|   Microchip Technology Inc.
|   PolarFire IBIS Model
[IBIS ver]   5.0
[File name]   polarfire_gpio_diff.ibs
[File Rev]   2.4
[Date]   Fri Nov 24 2023
[Source] Simulated Models ONLY.
   All data is based on Spice simulation. All performed at Microchip Technology Inc.
[Notes]   This IBIS file is for GPIO Differential Standards.
   Please refer to polarfire_gpio_se.ibs for GPIO single ended Standards Configurations,
   and refer to polarfire_hsio_se.ibs and polarfire_hsio_diff.ibs for HSIO Configurations.
   The package parasitics of various package types are given.
   Uncomment the appropriate package before simulations
   Revision History
   Rev 2.4: 24-Nov-2023
   - Added clamp-off configuration support for LCMDS25,SLVS25,LVDS25,PPDS25,RSDS25,SUBLVDS25,
   MINILVDS25,HCSL25 receivers
   - Added mixed mode receiver support for HSUL18_33_ODT-OFF,HSUL18_25_ODT-OFF,HSUL18_15_ODT-OFF,
   HSUL18_12_ODT-OFF,HSUL18_ODT-OFF,HSUL18_ODT-50
   - Updated Vinl and Vinh values of HCSL33, HCSL25 receivers
   Rev 2.3: 20-Jun-2023
   - Added VCM-LOW configuration support for SLVS33,SLVS25,LVDS33,LVDS25,RSDS33,RSDS25,
   MINILVDS33,MINILVDS25,SUBLVDS33,SUBLVDS25,PPDS33,PPDS25,HCSL33,HCSL25,LVPECL33,LVDS18G receivers
   - Updated Vmeas values of LCMDS33,LCMDS25,MIPIE25 drivers
   - Updated Vinl and Vinh values of SLVS33,SLVS25 receivers
   Rev 2.2: 4-May-2022
   - Added MPF050 device with RLC package data in [Package] section
   - Added RLC package type of FCG784N for MPF300T/TS device
   - Update RLC values of 200T-FCVG484 device package data
   Rev 2.1: 06-Sept-2021
   - Added support for LVDS18G driver and receiver
   - All LVDS type differential driver models updated to provide stable common mode voltage
[Disclaimer] This information is for board design considerations.
   Simulation based V/I curves contained in this model file are
   considered preliminary until verified against bench
   measurements. Maximum currents may vary from part to part but
   should not exceed maximum I/V curves provided in this model file.
[Copyright]  (c) 2023, Microchip Technology Inc., All Rights Reserved.
| ADDITIONAL NOTES
|For High Speed Mobile Industry Processor Interface (MIPI) configuration,please use LVDS25 receiver IBIS models.
|Warnings for ISSO Pullup, Pulldown currents being non-zero maybe ignored.
|Cautions for Ramp data maybe ignored.
|The naming conventions used in the signal_name/model_name are as follows:
| SLEW-#  - Slew setting,OFF or ON represented by #
| HYST-# and HYS-#  - Hysteresis setting,OFF or ON represented by #
| #mA   - Driver current strength, value represented by #
| #ohm   - Driver impedance mode, value represented by #
| ODT-# and OD-#   - Series on-die termination, impedance value represented by #
| CL   - Receiver standards with clamp ON
| C1   - Refers to Class-I driver models
| C2   - Refers to Class-II driver models
| #_I   - Refers to input models ,  model name represented by #
| #_O   - Refers to output models , model name represented by #
| VCML   - Refers to LOW Vcm setting
| VCMM   - Refers to MID Vcm setting
| IBIS MODEL CHECKLIST
| Microchip Technology Inc. is dedicated to releasing quality IBIS models to customers.
| The following items have been
| verified for this IBIS model before release:
| 1)  Checked IBIS model by the golden parser ibischk5 [Complete]
| 2)  Ensured no errors reported by golden parser
|   for the IBIS model [Complete]
| 3)  Defined Vinl and Vinh for receivers [Complete]
| 4)  Defined Standard Load and Vmeas values for drivers [Complete]
| 5)  Defined overshoots for drivers and receivers [NA]
| 6)  Validated Ramp Values[]
| 7)  Defined V-T Tables for all output drivers [Complete]
| 8)  Validated [Diff Pins] [Complete]
| 9)  Verified Package Parasitics [Complete]
| 10) Defined Standard Load Parameters and Specifications
|   for waveforms [Complete]
| 11) Defined and Validate Pin mappings [Complete]
| 12) Verified C_comp_pullup and C_comp_pulldown Values []
| 13) Visually Inspected I-V Curves and V-T Tables  [Complete]
| 14) Presented Typ/Min/Max Values in the correct order for
|   all tables and parameters [Complete]
| 15) Simulated all output models with standard load and
|   switching through Vmeas [Complete]
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[Component]   PolarFire
[Manufacturer]   Microchip Technology Inc
[Package]
|   typ   min   max
|MPF050T/TL/TLS/TS
|R_pkg   0.342   NA   NA   | MPF050T/TL/TLS/TS-FCSG325
|L_pkg   2.917nH   NA   NA   | MPF050T/TL/TLS/TS-FCSG325
|C_pkg   1.401pF   NA   NA   | MPF050T/TL/TLS/TS-FCSG325
|R_pkg   0.668   NA   NA   | MPF050T/TL/TLS/TS-FCVG484
|L_pkg   4.858nH   NA   NA   | MPF050T/TL/TLS/TS-FCVG484
|C_pkg   1.717pF   NA   NA   | MPF050T/TL/TLS/TS-FCVG484
|MPF100T/TL/TLS/TS
|R_pkg   0.277   NA   NA   | MPF100T/TL/TLS/TS-FCSG325
|L_pkg   2.866nH   NA   NA   | MPF100T/TL/TLS/TS-FCSG325
|C_pkg   0.601pF   NA   NA   | MPF100T/TL/TLS/TS-FCSG325
|R_pkg   0.960   NA   NA   | MPF100T/TL/TLS/TS-FCG484
|L_pkg   6.090nH   NA   NA   | MPF100T/TL/TLS/TS-FCG484
|C_pkg   2.182pF   NA   NA   | MPF100T/TL/TLS/TS-FCG484
|R_pkg   0.639   NA   NA   | MPF100T/TL/TLS/TS-FCVG484
|L_pkg   4.241nH   NA   NA   | MPF100T/TL/TLS/TS-FCVG484
|C_pkg   1.595pF   NA   NA   | MPF100T/TL/TLS/TS-FCVG484
|MPF200T/TL/TLS/TS
|R_pkg   0.392   NA   NA   | MPF200T/TL/TLS/TS-FCSG325
|L_pkg   3.035nH   NA   NA   | MPF200T/TL/TLS/TS-FCSG325
|C_pkg   0.970pF   NA   NA   | MPF200T/TL/TLS/TS-FCSG325
|R_pkg   0.885   NA   NA   | MPF200T/TL/TLS/TS-FCG484
|L_pkg   5.836nH   NA   NA   | MPF200T/TL/TLS/TS-FCG484
|C_pkg   2.013pF   NA   NA   | MPF200T/TL/TLS/TS-FCG484
|R_pkg   0.634   NA   NA   | MPF200T/TL/TLS/TS-FCVG484
|L_pkg   4.221nH   NA   NA   | MPF200T/TL/TLS/TS-FCVG484
|C_pkg   1.605pF   NA   NA   | MPF200T/TL/TLS/TS-FCVG484
|R_pkg   0.483   NA   NA   | MPF200T/TL/TLS/TS-FCSG536
|L_pkg   4.073nH   NA   NA   | MPF200T/TL/TLS/TS-FCSG536
|C_pkg   1.335pF   NA   NA   | MPF200T/TL/TLS/TS-FCSG536
|R_pkg   1.512   NA   NA   | MPF200T/TL/TLS/TS-FCG784
|L_pkg   9.182nH   NA   NA   | MPF200T/TL/TLS/TS-FCG784
|C_pkg   3.029pF   NA   NA   | MPF200T/TL/TLS/TS-FCG784
|MPF300T/TL/TLS/TS
|R_pkg   0.678   NA   NA   | MPF300T/TL/TLS/TS-FCG484
|L_pkg   5.038nH   NA   NA   | MPF300T/TL/TLS/TS-FCG484
|C_pkg   1.584pF   NA   NA   | MPF300T/TL/TLS/TS-FCG484
|R_pkg   0.702   NA   NA   | MPF300T/TL/TLS/TS-FCVG484
|L_pkg   4.503nH   NA   NA   | MPF300T/TL/TLS/TS-FCVG484
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R_pkg   1.478   NA   NA   | MPF300T/TL/TLS/TS-FCG1152
L_pkg   8.879nH   NA   NA   | MPF300T/TL/TLS/TS-FCG1152
C_pkg   2.839pF   NA   NA   | MPF300T/TL/TLS/TS-FCG1152
|MPF500T/TL/TLS/TS
|R_pkg   1.081   NA   NA   | MPF500T/TL/TLS/TS-FCG784
|L_pkg   6.727nH   NA   NA   | MPF500T/TL/TLS/TS-FCG784
|C_pkg   2.413pF   NA   NA   | MPF500T/TL/TLS/TS-FCG784
|R_pkg   1.419   NA   NA   | MPF500T/TL/TLS/TS-FCG1152
|L_pkg   8.917nH   NA   NA   | MPF500T/TL/TLS/TS-FCG1152
|C_pkg   2.924pF   NA   NA   | MPF500T/TL/TLS/TS-FCG1152
| End Header
| The PIN numbers given below are examples. They do not correspond to
| device pin numbers.
[Pin]   signal_name   model_name   R_pin   L_pin   C_pin
1N   SSTL25D_C1_80ohm_SLEW-OFF_N_O   SSTL25_C1_80ohm_SLEW-OFF_GPIO_O
1P   SSTL25D_C1_80ohm_SLEW-OFF_P_O   SSTL25_C1_80ohm_SLEW-OFF_GPIO_O
2N   SSTL25D_C1_120ohm_SLEW-OFF_N_O   SSTL25_C1_120ohm_SLEW-OFF_GPIO_O
2P   SSTL25D_C1_120ohm_SLEW-OFF_P_O   SSTL25_C1_120ohm_SLEW-OFF_GPIO_O
3N   SSTL25D_C1_60ohm_SLEW-OFF_N_O   SSTL25_C1_60ohm_SLEW-OFF_GPIO_O
3P   SSTL25D_C1_60ohm_SLEW-OFF_P_O   SSTL25_C1_60ohm_SLEW-OFF_GPIO_O
4N   SSTL25D_C1_48ohm_SLEW-OFF_N_O   SSTL25_C1_48ohm_SLEW-OFF_GPIO_O
4P   SSTL25D_C1_48ohm_SLEW-OFF_P_O   SSTL25_C1_48ohm_SLEW-OFF_GPIO_O
5N   SSTL25D_C2_48ohm_SLEW-OFF_N_O   SSTL25_C2_48ohm_SLEW-OFF_GPIO_O
5P   SSTL25D_C2_48ohm_SLEW-OFF_P_O   SSTL25_C2_48ohm_SLEW-OFF_GPIO_O
6N   SSTL25D_C2_60ohm_SLEW-OFF_N_O   SSTL25_C2_60ohm_SLEW-OFF_GPIO_O
6P   SSTL25D_C2_60ohm_SLEW-OFF_P_O   SSTL25_C2_60ohm_SLEW-OFF_GPIO_O
7N   SSTL25D_C2_40ohm_SLEW-OFF_N_O   SSTL25_C2_40ohm_SLEW-OFF_GPIO_O
7P   SSTL25D_C2_40ohm_SLEW-OFF_P_O   SSTL25_C2_40ohm_SLEW-OFF_GPIO_O
8N   SSTL25D_C2_34ohm_SLEW-OFF_N_O   SSTL25_C2_34ohm_SLEW-OFF_GPIO_O
8P   SSTL25D_C2_34ohm_SLEW-OFF_P_O   SSTL25_C2_34ohm_SLEW-OFF_GPIO_O
9N   SSTL18D_C1_60ohm_SLEW-OFF_N_O   SSTL18_C1_60ohm_SLEW-OFF_GPIO_O
9P   SSTL18D_C1_60ohm_SLEW-OFF_P_O   SSTL18_C1_60ohm_SLEW-OFF_GPIO_O
10N   SSTL18D_C1_80ohm_SLEW-OFF_N_O   SSTL18_C1_80ohm_SLEW-OFF_GPIO_O
10P   SSTL18D_C1_80ohm_SLEW-OFF_P_O   SSTL18_C1_80ohm_SLEW-OFF_GPIO_O
11N   SSTL18D_C1_48ohm_SLEW-OFF_N_O   SSTL18_C1_48ohm_SLEW-OFF_GPIO_O
11P   SSTL18D_C1_48ohm_SLEW-OFF_P_O   SSTL18_C1_48ohm_SLEW-OFF_GPIO_O
12N   SSTL18D_C1_40ohm_SLEW-OFF_N_O   SSTL18_C1_40ohm_SLEW-OFF_GPIO_O
12P   SSTL18D_C1_40ohm_SLEW-OFF_P_O   SSTL18_C1_40ohm_SLEW-OFF_GPIO_O
13N   SSTL18D_C2_40ohm_SLEW-OFF_N_O   SSTL18_C2_40ohm_SLEW-OFF_GPIO_O
13P   SSTL18D_C2_40ohm_SLEW-OFF_P_O   SSTL18_C2_40ohm_SLEW-OFF_GPIO_O
14N   SSTL18D_C2_48ohm_SLEW-OFF_N_O   SSTL18_C2_48ohm_SLEW-OFF_GPIO_O
14P   SSTL18D_C2_48ohm_SLEW-OFF_P_O   SSTL18_C2_48ohm_SLEW-OFF_GPIO_O
15N   SSTL18D_C2_34ohm_SLEW-OFF_N_O   SSTL18_C2_34ohm_SLEW-OFF_GPIO_O
15P   SSTL18D_C2_34ohm_SLEW-OFF_P_O   SSTL18_C2_34ohm_SLEW-OFF_GPIO_O
16N   SSTL18D_C2_30ohm_SLEW-OFF_N_O   SSTL18_C2_30ohm_SLEW-OFF_GPIO_O
16P   SSTL18D_C2_30ohm_SLEW-OFF_P_O   SSTL18_C2_30ohm_SLEW-OFF_GPIO_O
17N   SSTL15D_C1_40ohm_SLEW-OFF_N_O   SSTL15_C1_40ohm_SLEW-OFF_GPIO_O
17P   SSTL15D_C1_40ohm_SLEW-OFF_P_O   SSTL15_C1_40ohm_SLEW-OFF_GPIO_O
18N   SSTL15D_C1_48ohm_SLEW-OFF_N_O   SSTL15_C1_48ohm_SLEW-OFF_GPIO_O
18P   SSTL15D_C1_48ohm_SLEW-OFF_P_O   SSTL15_C1_48ohm_SLEW-OFF_GPIO_O
19N   SSTL15D_C2_34ohm_SLEW-OFF_N_O   SSTL15_C2_34ohm_SLEW-OFF_GPIO_O
19P   SSTL15D_C2_34ohm_SLEW-OFF_P_O   SSTL15_C2_34ohm_SLEW-OFF_GPIO_O
20N   SSTL15D_C2_30ohm_SLEW-OFF_N_O   SSTL15_C2_30ohm_SLEW-OFF_GPIO_O
20P   SSTL15D_C2_30ohm_SLEW-OFF_P_O   SSTL15_C2_30ohm_SLEW-OFF_GPIO_O
21N   SSTL15D_C2_27ohm_SLEW-OFF_N_O   SSTL15_C2_27ohm_SLEW-OFF_GPIO_O
21P   SSTL15D_C2_27ohm_SLEW-OFF_P_O   SSTL15_C2_27ohm_SLEW-OFF_GPIO_O
22N   HSUL18D_C1_55ohm_SLEW-OFF_N_O   HSUL18_C1_55ohm_SLEW-OFF_GPIO_O
22P   HSUL18D_C1_55ohm_SLEW-OFF_P_O   HSUL18_C1_55ohm_SLEW-OFF_GPIO_O
23N   HSUL18D_C1_60ohm_SLEW-OFF_N_O   HSUL18_C1_60ohm_SLEW-OFF_GPIO_O
23P   HSUL18D_C1_60ohm_SLEW-OFF_P_O   HSUL18_C1_60ohm_SLEW-OFF_GPIO_O
24N   HSUL18D_C1_40ohm_SLEW-OFF_N_O   HSUL18_C1_40ohm_SLEW-OFF_GPIO_O
24P   HSUL18D_C1_40ohm_SLEW-OFF_P_O   HSUL18_C1_40ohm_SLEW-OFF_GPIO_O
25N   HSUL18D_C1_34ohm_SLEW-OFF_N_O   HSUL18_C1_34ohm_SLEW-OFF_GPIO_O
25P   HSUL18D_C1_34ohm_SLEW-OFF_P_O   HSUL18_C1_34ohm_SLEW-OFF_GPIO_O
26N   HSUL18D_C2_25ohm_SLEW-OFF_N_O   HSUL18_C2_25ohm_SLEW-OFF_GPIO_O
26P   HSUL18D_C2_25ohm_SLEW-OFF_P_O   HSUL18_C2_25ohm_SLEW-OFF_GPIO_O
27N   HSUL18D_C2_30ohm_SLEW-OFF_N_O   HSUL18_C2_30ohm_SLEW-OFF_GPIO_O
27P   HSUL18D_C2_30ohm_SLEW-OFF_P_O   HSUL18_C2_30ohm_SLEW-OFF_GPIO_O
28N   HSUL18D_C2_27ohm_SLEW-OFF_N_O   HSUL18_C2_27ohm_SLEW-OFF_GPIO_O
28P   HSUL18D_C2_27ohm_SLEW-OFF_P_O   HSUL18_C2_27ohm_SLEW-OFF_GPIO_O
29N   HSUL18D_C2_22ohm_SLEW-OFF_N_O   HSUL18_C2_22ohm_SLEW-OFF_GPIO_O
29P   HSUL18D_C2_22ohm_SLEW-OFF_P_O   HSUL18_C2_22ohm_SLEW-OFF_GPIO_O
30N   HSTL15D_C1_50ohm_SLEW-OFF_N_O   HSTL15_C1_50ohm_SLEW-OFF_GPIO_O
30P   HSTL15D_C1_50ohm_SLEW-OFF_P_O   HSTL15_C1_50ohm_SLEW-OFF_GPIO_O
31N   HSTL15D_C1_60ohm_SLEW-OFF_N_O   HSTL15_C1_60ohm_SLEW-OFF_GPIO_O
31P   HSTL15D_C1_60ohm_SLEW-OFF_P_O   HSTL15_C1_60ohm_SLEW-OFF_GPIO_O
32N   HSTL15D_C1_40ohm_SLEW-OFF_N_O   HSTL15_C1_40ohm_SLEW-OFF_GPIO_O
32P   HSTL15D_C1_40ohm_SLEW-OFF_P_O   HSTL15_C1_40ohm_SLEW-OFF_GPIO_O
33N   HSTL15D_C1_34ohm_SLEW-OFF_N_O   HSTL15_C1_34ohm_SLEW-OFF_GPIO_O
33P   HSTL15D_C1_34ohm_SLEW-OFF_P_O   HSTL15_C1_34ohm_SLEW-OFF_GPIO_O
34N   HSTL15D_C2_25ohm_SLEW-OFF_N_O   HSTL15_C2_25ohm_SLEW-OFF_GPIO_O
34P   HSTL15D_C2_25ohm_SLEW-OFF_P_O   HSTL15_C2_25ohm_SLEW-OFF_GPIO_O
35N   HSTL15D_C2_30ohm_SLEW-OFF_N_O   HSTL15_C2_30ohm_SLEW-OFF_GPIO_O
35P   HSTL15D_C2_30ohm_SLEW-OFF_P_O   HSTL15_C2_30ohm_SLEW-OFF_GPIO_O
36N   HSTL15D_C2_27ohm_SLEW-OFF_N_O   HSTL15_C2_27ohm_SLEW-OFF_GPIO_O
36P   HSTL15D_C2_27ohm_SLEW-OFF_P_O   HSTL15_C2_27ohm_SLEW-OFF_GPIO_O
37N   HSTL15D_C2_22ohm_SLEW-OFF_N_O   HSTL15_C2_22ohm_SLEW-OFF_GPIO_O
37P   HSTL15D_C2_22ohm_SLEW-OFF_P_O   HSTL15_C2_22ohm_SLEW-OFF_GPIO_O
38N   LVCMOS33D_8mA_SLEW-ON_N_O   LVCMOS33_8mA_SLEW-ON_GPIO_O
38P   LVCMOS33D_8mA_SLEW-ON_P_O   LVCMOS33_8mA_SLEW-ON_GPIO_O
39N   LVCMOS33D_8mA_SLEW-OFF_N_O   LVCMOS33_8mA_SLEW-OFF_GPIO_O
39P   LVCMOS33D_8mA_SLEW-OFF_P_O   LVCMOS33_8mA_SLEW-OFF_GPIO_O
40N   LVCMOS33D_2mA_SLEW-ON_N_O   LVCMOS33_2mA_SLEW-ON_GPIO_O
40P   LVCMOS33D_2mA_SLEW-ON_P_O   LVCMOS33_2mA_SLEW-ON_GPIO_O
41N   LVCMOS33D_2mA_SLEW-OFF_N_O   LVCMOS33_2mA_SLEW-OFF_GPIO_O
41P   LVCMOS33D_2mA_SLEW-OFF_P_O   LVCMOS33_2mA_SLEW-OFF_GPIO_O
42N   LVCMOS33D_4mA_SLEW-ON_N_O   LVCMOS33_4mA_SLEW-ON_GPIO_O
42P   LVCMOS33D_4mA_SLEW-ON_P_O   LVCMOS33_4mA_SLEW-ON_GPIO_O
43N   LVCMOS33D_4mA_SLEW-OFF_N_O   LVCMOS33_4mA_SLEW-OFF_GPIO_O
43P   LVCMOS33D_4mA_SLEW-OFF_P_O   LVCMOS33_4mA_SLEW-OFF_GPIO_O
44N   LVCMOS33D_12mA_SLEW-ON_N_O   LVCMOS33_12mA_SLEW-ON_GPIO_O
44P   LVCMOS33D_12mA_SLEW-ON_P_O   LVCMOS33_12mA_SLEW-ON_GPIO_O
45N   LVCMOS33D_12mA_SLEW-OFF_N_O   LVCMOS33_12mA_SLEW-OFF_GPIO_O
45P   LVCMOS33D_12mA_SLEW-OFF_P_O   LVCMOS33_12mA_SLEW-OFF_GPIO_O
46N   LVCMOS33D_16mA_SLEW-ON_N_O   LVCMOS33_16mA_SLEW-ON_GPIO_O
46P   LVCMOS33D_16mA_SLEW-ON_P_O   LVCMOS33_16mA_SLEW-ON_GPIO_O
47N   LVCMOS33D_16mA_SLEW-OFF_N_O   LVCMOS33_16mA_SLEW-OFF_GPIO_O
47P   LVCMOS33D_16mA_SLEW-OFF_P_O   LVCMOS33_16mA_SLEW-OFF_GPIO_O
48N   LVCMOS33D_20mA_SLEW-ON_N_O   LVCMOS33_20mA_SLEW-ON_GPIO_O
48P   LVCMOS33D_20mA_SLEW-ON_P_O   LVCMOS33_20mA_SLEW-ON_GPIO_O
49N   LVCMOS33D_20mA_SLEW-OFF_N_O   LVCMOS33_20mA_SLEW-OFF_GPIO_O
49P   LVCMOS33D_20mA_SLEW-OFF_P_O   LVCMOS33_20mA_SLEW-OFF_GPIO_O
50N   LVCMOS25D_8mA_SLEW-ON_N_O   LVCMOS25_8mA_SLEW-ON_GPIO_O
50P   LVCMOS25D_8mA_SLEW-ON_P_O   LVCMOS25_8mA_SLEW-ON_GPIO_O
51N   LVCMOS25D_8mA_SLEW-OFF_N_O   LVCMOS25_8mA_SLEW-OFF_GPIO_O
51P   LVCMOS25D_8mA_SLEW-OFF_P_O   LVCMOS25_8mA_SLEW-OFF_GPIO_O
52N   LVCMOS25D_2mA_SLEW-ON_N_O   LVCMOS25_2mA_SLEW-ON_GPIO_O
52P   LVCMOS25D_2mA_SLEW-ON_P_O   LVCMOS25_2mA_SLEW-ON_GPIO_O
53N   LVCMOS25D_2mA_SLEW-OFF_N_O   LVCMOS25_2mA_SLEW-OFF_GPIO_O
53P   LVCMOS25D_2mA_SLEW-OFF_P_O   LVCMOS25_2mA_SLEW-OFF_GPIO_O
54N   LVCMOS25D_4mA_SLEW-ON_N_O   LVCMOS25_4mA_SLEW-ON_GPIO_O
54P   LVCMOS25D_4mA_SLEW-ON_P_O   LVCMOS25_4mA_SLEW-ON_GPIO_O
55N   LVCMOS25D_4mA_SLEW-OFF_N_O   LVCMOS25_4mA_SLEW-OFF_GPIO_O
55P   LVCMOS25D_4mA_SLEW-OFF_P_O   LVCMOS25_4mA_SLEW-OFF_GPIO_O
56N   LVCMOS25D_6mA_SLEW-ON_N_O   LVCMOS25_6mA_SLEW-ON_GPIO_O
56P   LVCMOS25D_6mA_SLEW-ON_P_O   LVCMOS25_6mA_SLEW-ON_GPIO_O
57N   LVCMOS25D_6mA_SLEW-OFF_N_O   LVCMOS25_6mA_SLEW-OFF_GPIO_O
57P   LVCMOS25D_6mA_SLEW-OFF_P_O   LVCMOS25_6mA_SLEW-OFF_GPIO_O
58N   LVCMOS25D_12mA_SLEW-ON_N_O   LVCMOS25_12mA_SLEW-ON_GPIO_O
58P   LVCMOS25D_12mA_SLEW-ON_P_O   LVCMOS25_12mA_SLEW-ON_GPIO_O
59N   LVCMOS25D_12mA_SLEW-OFF_N_O   LVCMOS25_12mA_SLEW-OFF_GPIO_O
59P   LVCMOS25D_12mA_SLEW-OFF_P_O   LVCMOS25_12mA_SLEW-OFF_GPIO_O
60N   LVCMOS25D_16mA_SLEW-ON_N_O   LVCMOS25_16mA_SLEW-ON_GPIO_O
60P   LVCMOS25D_16mA_SLEW-ON_P_O   LVCMOS25_16mA_SLEW-ON_GPIO_O
61N   LVCMOS25D_16mA_SLEW-OFF_N_O   LVCMOS25_16mA_SLEW-OFF_GPIO_O
61P   LVCMOS25D_16mA_SLEW-OFF_P_O   LVCMOS25_16mA_SLEW-OFF_GPIO_O
62N   LVCMOS18D_8mA_SLEW-OFF_N_O   LVCMOS18_8mA_SLEW-OFF_GPIO_O
62P   LVCMOS18D_8mA_SLEW-OFF_P_O   LVCMOS18_8mA_SLEW-OFF_GPIO_O
63N   LVCMOS18D_2mA_SLEW-OFF_N_O   LVCMOS18_2mA_SLEW-OFF_GPIO_O
63P   LVCMOS18D_2mA_SLEW-OFF_P_O   LVCMOS18_2mA_SLEW-OFF_GPIO_O
64N   LVCMOS18D_4mA_SLEW-OFF_N_O   LVCMOS18_4mA_SLEW-OFF_GPIO_O
64P   LVCMOS18D_4mA_SLEW-OFF_P_O   LVCMOS18_4mA_SLEW-OFF_GPIO_O
65N   LVCMOS18D_6mA_SLEW-OFF_N_O   LVCMOS18_6mA_SLEW-OFF_GPIO_O
65P   LVCMOS18D_6mA_SLEW-OFF_P_O   LVCMOS18_6mA_SLEW-OFF_GPIO_O
66N   LVCMOS18D_10mA_SLEW-OFF_N_O   LVCMOS18_10mA_SLEW-OFF_GPIO_O
66P   LVCMOS18D_10mA_SLEW-OFF_P_O   LVCMOS18_10mA_SLEW-OFF_GPIO_O
67N   LVCMOS18D_12mA_SLEW-OFF_N_O   LVCMOS18_12mA_SLEW-OFF_GPIO_O
67P   LVCMOS18D_12mA_SLEW-OFF_P_O   LVCMOS18_12mA_SLEW-OFF_GPIO_O
68N   LVCMOS15D_8mA_SLEW-OFF_N_O   LVCMOS15_8mA_SLEW-OFF_GPIO_O
68P   LVCMOS15D_8mA_SLEW-OFF_P_O   LVCMOS15_8mA_SLEW-OFF_GPIO_O
69N   LVCMOS15D_2mA_SLEW-OFF_N_O   LVCMOS15_2mA_SLEW-OFF_GPIO_O
69P   LVCMOS15D_2mA_SLEW-OFF_P_O   LVCMOS15_2mA_SLEW-OFF_GPIO_O
70N   LVCMOS15D_4mA_SLEW-OFF_N_O   LVCMOS15_4mA_SLEW-OFF_GPIO_O
70P   LVCMOS15D_4mA_SLEW-OFF_P_O   LVCMOS15_4mA_SLEW-OFF_GPIO_O
71N   LVCMOS15D_6mA_SLEW-OFF_N_O   LVCMOS15_6mA_SLEW-OFF_GPIO_O
71P   LVCMOS15D_6mA_SLEW-OFF_P_O   LVCMOS15_6mA_SLEW-OFF_GPIO_O
72N   LVCMOS15D_10mA_SLEW-OFF_N_O   LVCMOS15_10mA_SLEW-OFF_GPIO_O
72P   LVCMOS15D_10mA_SLEW-OFF_P_O   LVCMOS15_10mA_SLEW-OFF_GPIO_O
73N   LVCMOS12D_8mA_SLEW-OFF_N_O   LVCMOS12_8mA_SLEW-OFF_GPIO_O
73P   LVCMOS12D_8mA_SLEW-OFF_P_O   LVCMOS12_8mA_SLEW-OFF_GPIO_O
74N   LVCMOS12D_2mA_SLEW-OFF_N_O   LVCMOS12_2mA_SLEW-OFF_GPIO_O
74P   LVCMOS12D_2mA_SLEW-OFF_P_O   LVCMOS12_2mA_SLEW-OFF_GPIO_O
75N   LVCMOS12D_4mA_SLEW-OFF_N_O   LVCMOS12_4mA_SLEW-OFF_GPIO_O
75P   LVCMOS12D_4mA_SLEW-OFF_P_O   LVCMOS12_4mA_SLEW-OFF_GPIO_O
76N   LVCMOS12D_6mA_SLEW-OFF_N_O   LVCMOS12_6mA_SLEW-OFF_GPIO_O
76P   LVCMOS12D_6mA_SLEW-OFF_P_O   LVCMOS12_6mA_SLEW-OFF_GPIO_O
77N   SLVS33_CL_ODT-OFF_HYST-OFF_N_I   SLVS33_CL_ODT-OFF_HYST-OFF_GPIO_I
77P   SLVS33_CL_ODT-OFF_HYST-OFF_P_I   SLVS33_CL_ODT-OFF_HYST-OFF_GPIO_I
78N   SLVS25_CL_ODT-OFF_HYST-OFF_N_I   SLVS25_CL_ODT-OFF_HYST-OFF_GPIO_I
78P   SLVS25_CL_ODT-OFF_HYST-OFF_P_I   SLVS25_CL_ODT-OFF_HYST-OFF_GPIO_I
79N   SSTL25D_33_CL_ODT-OFF_HYST-OFF_N_I   SSTL25_33_CL_ODT-OFF_HYST-OFF_GPIO_N_I
79P   SSTL25D_33_CL_ODT-OFF_HYST-OFF_P_I   SSTL25_33_CL_ODT-OFF_HYST-OFF_GPIO_P_I
80N   SSTL25D_33_CL_ODT-100_HYST-OFF_N_I   SSTL25_33_CL_ODT-OFF_HYST-OFF_GPIO_N_I
80P   SSTL25D_33_CL_ODT-100_HYST-OFF_P_I   SSTL25_33_CL_ODT-OFF_HYST-OFF_GPIO_P_I
81N   SSTL25D_CL_ODT-OFF_HYST-OFF_N_I   SSTL25_CL_ODT-OFF_HYST-OFF_GPIO_N_I
81P   SSTL25D_CL_ODT-OFF_HYST-OFF_P_I   SSTL25_CL_ODT-OFF_HYST-OFF_GPIO_P_I
82N   SSTL25D_CL_ODT-100_HYST-OFF_N_I   SSTL25_CL_ODT-OFF_HYST-OFF_GPIO_N_I
82P   SSTL25D_CL_ODT-100_HYST-OFF_P_I   SSTL25_CL_ODT-OFF_HYST-OFF_GPIO_P_I
83N   SSTL25D_33_ODT-OFF_HYST-OFF_N_I   SSTL25_33_ODT-OFF_HYST-OFF_GPIO_N_I
83P   SSTL25D_33_ODT-OFF_HYST-OFF_P_I   SSTL25_33_ODT-OFF_HYST-OFF_GPIO_P_I
84N   SSTL25D_ODT-OFF_HYST-OFF_N_I   SSTL25_ODT-OFF_HYST-OFF_GPIO_N_I
84P   SSTL25D_ODT-OFF_HYST-OFF_P_I   SSTL25_ODT-OFF_HYST-OFF_GPIO_P_I
85N   SSTL25D_18_ODT-OFF_HYST-OFF_N_I   SSTL25_18_ODT-OFF_HYST-OFF_GPIO_N_I
85P   SSTL25D_18_ODT-OFF_HYST-OFF_P_I   SSTL25_18_ODT-OFF_HYST-OFF_GPIO_P_I
86N   SSTL25D_15_ODT-OFF_HYST-OFF_N_I   SSTL25_15_ODT-OFF_HYST-OFF_GPIO_N_I
86P   SSTL25D_15_ODT-OFF_HYST-OFF_P_I   SSTL25_15_ODT-OFF_HYST-OFF_GPIO_P_I
87N   SSTL25D_12_ODT-OFF_HYST-OFF_N_I   SSTL25_12_ODT-OFF_HYST-OFF_GPIO_N_I
87P   SSTL25D_12_ODT-OFF_HYST-OFF_P_I   SSTL25_12_ODT-OFF_HYST-OFF_GPIO_P_I
88N   SSTL25D_33_ODT-100_HYST-OFF_N_I   SSTL25_33_ODT-OFF_HYST-OFF_GPIO_N_I
88P   SSTL25D_33_ODT-100_HYST-OFF_P_I   SSTL25_33_ODT-OFF_HYST-OFF_GPIO_P_I
89N   SSTL25D_ODT-100_HYST-OFF_N_I   SSTL25_ODT-OFF_HYST-OFF_GPIO_N_I
89P   SSTL25D_ODT-100_HYST-OFF_P_I   SSTL25_ODT-OFF_HYST-OFF_GPIO_P_I
90N   SSTL25D_18_ODT-100_HYST-OFF_N_I   SSTL25_18_ODT-OFF_HYST-OFF_GPIO_N_I
90P   SSTL25D_18_ODT-100_HYST-OFF_P_I   SSTL25_18_ODT-OFF_HYST-OFF_GPIO_P_I
91N   SSTL25D_15_ODT-100_HYST-OFF_N_I   SSTL25_15_ODT-OFF_HYST-OFF_GPIO_N_I
91P   SSTL25D_15_ODT-100_HYST-OFF_P_I   SSTL25_15_ODT-OFF_HYST-OFF_GPIO_P_I
92N   SSTL25D_12_ODT-100_HYST-OFF_N_I   SSTL25_12_ODT-OFF_HYST-OFF_GPIO_N_I
92P   SSTL25D_12_ODT-100_HYST-OFF_P_I   SSTL25_12_ODT-OFF_HYST-OFF_GPIO_P_I
93N   SSTL18D_33_CL_ODT-OFF_HYST-OFF_N_I   SSTL18_33_CL_ODT-OFF_HYST-OFF_GPIO_I
93P   SSTL18D_33_CL_ODT-OFF_HYST-OFF_P_I   SSTL18_33_CL_ODT-OFF_HYST-OFF_GPIO_I
94N   SSTL18D_25_CL_ODT-OFF_HYST-OFF_N_I   SSTL18_25_CL_ODT-OFF_HYST-OFF_GPIO_I
94P   SSTL18D_25_CL_ODT-OFF_HYST-OFF_P_I   SSTL18_25_CL_ODT-OFF_HYST-OFF_GPIO_I
95N   SSTL18D_CL_ODT-OFF_HYST-OFF_N_I   SSTL18_CL_ODT-OFF_HYST-OFF_GPIO_I
95P   SSTL18D_CL_ODT-OFF_HYST-OFF_P_I   SSTL18_CL_ODT-OFF_HYST-OFF_GPIO_I
96N   SSTL18D_CL_ODT-50_HYST-OFF_N_I   SSTL18_CL_ODT-50_HYST-OFF_GPIO_I
96P   SSTL18D_CL_ODT-50_HYST-OFF_P_I   SSTL18_CL_ODT-50_HYST-OFF_GPIO_I
97N   SSTL18D_CL_ODT-150_HYST-OFF_N_I   SSTL18_CL_ODT-150_HYST-OFF_GPIO_I
97P   SSTL18D_CL_ODT-150_HYST-OFF_P_I   SSTL18_CL_ODT-150_HYST-OFF_GPIO_I
98N   SSTL18D_CL_ODT-75_HYST-OFF_N_I   SSTL18_CL_ODT-75_HYST-OFF_GPIO_I
98P   SSTL18D_CL_ODT-75_HYST-OFF_P_I   SSTL18_CL_ODT-75_HYST-OFF_GPIO_I
99N   SSTL18D_33_ODT-OFF_HYST-OFF_N_I   SSTL18_33_ODT-OFF_HYST-OFF_GPIO_I
99P   SSTL18D_33_ODT-OFF_HYST-OFF_P_I   SSTL18_33_ODT-OFF_HYST-OFF_GPIO_I
100N   SSTL18D_25_ODT-OFF_HYST-OFF_N_I   SSTL18_25_ODT-OFF_HYST-OFF_GPIO_I
100P   SSTL18D_25_ODT-OFF_HYST-OFF_P_I   SSTL18_25_ODT-OFF_HYST-OFF_GPIO_I
101N   SSTL18D_15_ODT-OFF_HYST-OFF_N_I   SSTL18_15_ODT-OFF_HYST-OFF_GPIO_I
101P   SSTL18D_15_ODT-OFF_HYST-OFF_P_I   SSTL18_15_ODT-OFF_HYST-OFF_GPIO_I
102N   SSTL18D_12_ODT-OFF_HYST-OFF_N_I   SSTL18_12_ODT-OFF_HYST-OFF_GPIO_I
102P   SSTL18D_12_ODT-OFF_HYST-OFF_P_I   SSTL18_12_ODT-OFF_HYST-OFF_GPIO_I
103N   SSTL18D_ODT-OFF_HYST-OFF_N_I   SSTL18_ODT-OFF_HYST-OFF_GPIO_I
103P   SSTL18D_ODT-OFF_HYST-OFF_P_I   SSTL18_ODT-OFF_HYST-OFF_GPIO_I
104N   SSTL18D_ODT-50_HYST-OFF_N_I   SSTL18_ODT-50_HYST-OFF_GPIO_I
104P   SSTL18D_ODT-50_HYST-OFF_P_I   SSTL18_ODT-50_HYST-OFF_GPIO_I
105N   SSTL18D_ODT-150_HYST-OFF_N_I   SSTL18_ODT-150_HYST-OFF_GPIO_I
105P   SSTL18D_ODT-150_HYST-OFF_P_I   SSTL18_ODT-150_HYST-OFF_GPIO_I
106N   SSTL18D_ODT-75_HYST-OFF_N_I   SSTL18_ODT-75_HYST-OFF_GPIO_I
106P   SSTL18D_ODT-75_HYST-OFF_P_I   SSTL18_ODT-75_HYST-OFF_GPIO_I
107N   SSTL15D_33_CL_ODT-OFF_HYST-OFF_N_I   SSTL15_33_CL_ODT-OFF_HYST-OFF_GPIO_I
107P   SSTL15D_33_CL_ODT-OFF_HYST-OFF_P_I   SSTL15_33_CL_ODT-OFF_HYST-OFF_GPIO_I
108N   SSTL15D_25_CL_ODT-OFF_HYST-OFF_N_I   SSTL15_25_CL_ODT-OFF_HYST-OFF_GPIO_I
108P   SSTL15D_25_CL_ODT-OFF_HYST-OFF_P_I   SSTL15_25_CL_ODT-OFF_HYST-OFF_GPIO_I
109N   SSTL15D_18_CL_ODT-OFF_HYST-OFF_N_I   SSTL15_18_CL_ODT-OFF_HYST-OFF_GPIO_I
109P   SSTL15D_18_CL_ODT-OFF_HYST-OFF_P_I   SSTL15_18_CL_ODT-OFF_HYST-OFF_GPIO_I
110N   SSTL15D_CL_ODT-OFF_HYST-OFF_N_I   SSTL15_CL_ODT-OFF_HYST-OFF_GPIO_I
110P   SSTL15D_CL_ODT-OFF_HYST-OFF_P_I   SSTL15_CL_ODT-OFF_HYST-OFF_GPIO_I
111N   SSTL15D_CL_ODT-60_HYST-OFF_N_I   SSTL15_CL_ODT-60_HYST-OFF_GPIO_I
111P   SSTL15D_CL_ODT-60_HYST-OFF_P_I   SSTL15_CL_ODT-60_HYST-OFF_GPIO_I
112N   SSTL15D_CL_ODT-120_HYST-OFF_N_I   SSTL15_CL_ODT-120_HYST-OFF_GPIO_I
112P   SSTL15D_CL_ODT-120_HYST-OFF_P_I   SSTL15_CL_ODT-120_HYST-OFF_GPIO_I
113N   SSTL15D_CL_ODT-40_HYST-OFF_N_I   SSTL15_CL_ODT-40_HYST-OFF_GPIO_I
113P   SSTL15D_CL_ODT-40_HYST-OFF_P_I   SSTL15_CL_ODT-40_HYST-OFF_GPIO_I
114N   SSTL15D_CL_ODT-30_HYST-OFF_N_I   SSTL15_CL_ODT-30_HYST-OFF_GPIO_I
114P   SSTL15D_CL_ODT-30_HYST-OFF_P_I   SSTL15_CL_ODT-30_HYST-OFF_GPIO_I
115N   SSTL15D_CL_ODT-20_HYST-OFF_N_I   SSTL15_CL_ODT-20_HYST-OFF_GPIO_I
115P   SSTL15D_CL_ODT-20_HYST-OFF_P_I   SSTL15_CL_ODT-20_HYST-OFF_GPIO_I
116N   SSTL15D_33_ODT-OFF_HYST-OFF_N_I   SSTL15_33_ODT-OFF_HYST-OFF_GPIO_I
116P   SSTL15D_33_ODT-OFF_HYST-OFF_P_I   SSTL15_33_ODT-OFF_HYST-OFF_GPIO_I
117N   SSTL15D_25_ODT-OFF_HYST-OFF_N_I   SSTL15_25_ODT-OFF_HYST-OFF_GPIO_I
117P   SSTL15D_25_ODT-OFF_HYST-OFF_P_I   SSTL15_25_ODT-OFF_HYST-OFF_GPIO_I
118N   SSTL15D_18_ODT-OFF_HYST-OFF_N_I   SSTL15_18_ODT-OFF_HYST-OFF_GPIO_I
118P   SSTL15D_18_ODT-OFF_HYST-OFF_P_I   SSTL15_18_ODT-OFF_HYST-OFF_GPIO_I
119N   SSTL15D_12_ODT-OFF_HYST-OFF_N_I   SSTL15_12_ODT-OFF_HYST-OFF_GPIO_I
119P   SSTL15D_12_ODT-OFF_HYST-OFF_P_I   SSTL15_12_ODT-OFF_HYST-OFF_GPIO_I
120N   SSTL15D_ODT-OFF_HYST-OFF_N_I   SSTL15_ODT-OFF_HYST-OFF_GPIO_I
120P   SSTL15D_ODT-OFF_HYST-OFF_P_I   SSTL15_ODT-OFF_HYST-OFF_GPIO_I
121N   SSTL15D_ODT-60_HYST-OFF_N_I   SSTL15_ODT-60_HYST-OFF_GPIO_I
121P   SSTL15D_ODT-60_HYST-OFF_P_I   SSTL15_ODT-60_HYST-OFF_GPIO_I
122N   SSTL15D_ODT-120_HYST-OFF_N_I   SSTL15_ODT-120_HYST-OFF_GPIO_I
122P   SSTL15D_ODT-120_HYST-OFF_P_I   SSTL15_ODT-120_HYST-OFF_GPIO_I
123N   SSTL15D_ODT-40_HYST-OFF_N_I   SSTL15_ODT-40_HYST-OFF_GPIO_I
123P   SSTL15D_ODT-40_HYST-OFF_P_I   SSTL15_ODT-40_HYST-OFF_GPIO_I
124N   SSTL15D_ODT-30_HYST-OFF_N_I   SSTL15_ODT-30_HYST-OFF_GPIO_I
124P   SSTL15D_ODT-30_HYST-OFF_P_I   SSTL15_ODT-30_HYST-OFF_GPIO_I
125N   SSTL15D_ODT-20_HYST-OFF_N_I   SSTL15_ODT-20_HYST-OFF_GPIO_I
125P   SSTL15D_ODT-20_HYST-OFF_P_I   SSTL15_ODT-20_HYST-OFF_GPIO_I
126N   HSUL18D_33_CL_ODT-OFF_HYST-OFF_N_I   HSUL18_33_CL_ODT-OFF_HYST-OFF_GPIO_I
126P   HSUL18D_33_CL_ODT-OFF_HYST-OFF_P_I   HSUL18_33_CL_ODT-OFF_HYST-OFF_GPIO_I
127N   HSUL18D_25_CL_ODT-OFF_HYST-OFF_N_I   HSUL18_25_CL_ODT-OFF_HYST-OFF_GPIO_I
127P   HSUL18D_25_CL_ODT-OFF_HYST-OFF_P_I   HSUL18_25_CL_ODT-OFF_HYST-OFF_GPIO_I
128N   HSUL18D_CL_ODT-OFF_HYST-OFF_N_I   HSUL18_CL_ODT-OFF_HYST-OFF_GPIO_I
128P   HSUL18D_CL_ODT-OFF_HYST-OFF_P_I   HSUL18_CL_ODT-OFF_HYST-OFF_GPIO_I
129N   HSUL18D_CL_ODT-50_HYST-OFF_N_I   HSUL18_CL_ODT-50_HYST-OFF_GPIO_I
129P   HSUL18D_CL_ODT-50_HYST-OFF_P_I   HSUL18_CL_ODT-50_HYST-OFF_GPIO_I
130N   HSTL15D_33_CL_ODT-OFF_HYST-OFF_N_I   HSTL15_33_CL_ODT-OFF_HYST-OFF_GPIO_I
130P   HSTL15D_33_CL_ODT-OFF_HYST-OFF_P_I   HSTL15_33_CL_ODT-OFF_HYST-OFF_GPIO_I
131N   HSTL15D_25_CL_ODT-OFF_HYST-OFF_N_I   HSTL15_25_CL_ODT-OFF_HYST-OFF_GPIO_I
131P   HSTL15D_25_CL_ODT-OFF_HYST-OFF_P_I   HSTL15_25_CL_ODT-OFF_HYST-OFF_GPIO_I
132N   HSTL15D_18_CL_ODT-OFF_HYST-OFF_N_I   HSTL15_18_CL_ODT-OFF_HYST-OFF_GPIO_I
132P   HSTL15D_18_CL_ODT-OFF_HYST-OFF_P_I   HSTL15_18_CL_ODT-OFF_HYST-OFF_GPIO_I
133N   HSTL15D_CL_ODT-OFF_HYST-OFF_N_I   HSTL15_CL_ODT-OFF_HYST-OFF_GPIO_I
133P   HSTL15D_CL_ODT-OFF_HYST-OFF_P_I   HSTL15_CL_ODT-OFF_HYST-OFF_GPIO_I
134N   HSTL15D_CL_ODT-50_HYST-OFF_N_I   HSTL15_CL_ODT-50_HYST-OFF_GPIO_I
134P   HSTL15D_CL_ODT-50_HYST-OFF_P_I   HSTL15_CL_ODT-50_HYST-OFF_GPIO_I
135N   HSTL15D_33_ODT-OFF_HYST-OFF_N_I   HSTL15_33_ODT-OFF_HYST-OFF_GPIO_I
135P   HSTL15D_33_ODT-OFF_HYST-OFF_P_I   HSTL15_33_ODT-OFF_HYST-OFF_GPIO_I
136N   HSTL15D_25_ODT-OFF_HYST-OFF_N_I   HSTL15_25_ODT-OFF_HYST-OFF_GPIO_I
136P   HSTL15D_25_ODT-OFF_HYST-OFF_P_I   HSTL15_25_ODT-OFF_HYST-OFF_GPIO_I
137N   HSTL15D_18_ODT-OFF_HYST-OFF_N_I   HSTL15_18_ODT-OFF_HYST-OFF_GPIO_I
137P   HSTL15D_18_ODT-OFF_HYST-OFF_P_I   HSTL15_18_ODT-OFF_HYST-OFF_GPIO_I
138N   HSTL15D_12_ODT-OFF_HYST-OFF_N_I   HSTL15_12_ODT-OFF_HYST-OFF_GPIO_I
138P   HSTL15D_12_ODT-OFF_HYST-OFF_P_I   HSTL15_12_ODT-OFF_HYST-OFF_GPIO_I
139N   HSTL15D_ODT-OFF_HYST-OFF_N_I   HSTL15_ODT-OFF_HYST-OFF_GPIO_I
139P   HSTL15D_ODT-OFF_HYST-OFF_P_I   HSTL15_ODT-OFF_HYST-OFF_GPIO_I
140N   HSTL15D_ODT-50_HYST-OFF_N_I   HSTL15_ODT-50_HYST-OFF_GPIO_I
140P   HSTL15D_ODT-50_HYST-OFF_P_I   HSTL15_ODT-50_HYST-OFF_GPIO_I
141N   LVDS33_6mA_SLEW-OFF_N_O   LVDS33_6mA_SLEW-OFF_GPIO_O
141P   LVDS33_6mA_SLEW-OFF_P_O   LVDS33_6mA_SLEW-OFF_GPIO_O
142N   LVDS33_6mA_SLEW-OFF_ODT-100_N_O   LVDS33_6mA_SLEW-OFF_GPIO_O
142P   LVDS33_6mA_SLEW-OFF_ODT-100_P_O   LVDS33_6mA_SLEW-OFF_GPIO_O
143N   LVDS33_4mA_SLEW-OFF_N_O   LVDS33_4mA_SLEW-OFF_GPIO_O
143P   LVDS33_4mA_SLEW-OFF_P_O   LVDS33_4mA_SLEW-OFF_GPIO_O
144N   LVDS33_4mA_SLEW-OFF_ODT-100_N_O   LVDS33_4mA_SLEW-OFF_GPIO_O
144P   LVDS33_4mA_SLEW-OFF_ODT-100_P_O   LVDS33_4mA_SLEW-OFF_GPIO_O
145N   LVDS33_3P5mA_SLEW-OFF_N_O   LVDS33_3P5mA_SLEW-OFF_GPIO_O
145P   LVDS33_3P5mA_SLEW-OFF_P_O   LVDS33_3P5mA_SLEW-OFF_GPIO_O
146N   LVDS33_3P5mA_SLEW-OFF_ODT-100_N_O   LVDS33_3P5mA_SLEW-OFF_GPIO_O
146P   LVDS33_3P5mA_SLEW-OFF_ODT-100_P_O   LVDS33_3P5mA_SLEW-OFF_GPIO_O
147N   LVDS33_3mA_SLEW-OFF_N_O   LVDS33_3mA_SLEW-OFF_GPIO_O
147P   LVDS33_3mA_SLEW-OFF_P_O   LVDS33_3mA_SLEW-OFF_GPIO_O
148N   LVDS33_3mA_SLEW-OFF_ODT-100_N_O   LVDS33_3mA_SLEW-OFF_GPIO_O
148P   LVDS33_3mA_SLEW-OFF_ODT-100_P_O   LVDS33_3mA_SLEW-OFF_GPIO_O
149N   LVDS25_6mA_SLEW-OFF_N_O   LVDS25_6mA_SLEW-OFF_GPIO_O
149P   LVDS25_6mA_SLEW-OFF_P_O   LVDS25_6mA_SLEW-OFF_GPIO_O
150N   LVDS25_6mA_SLEW-OFF_ODT-100_N_O   LVDS25_6mA_SLEW-OFF_GPIO_O
150P   LVDS25_6mA_SLEW-OFF_ODT-100_P_O   LVDS25_6mA_SLEW-OFF_GPIO_O
151N   LVDS25_4mA_SLEW-OFF_N_O   LVDS25_4mA_SLEW-OFF_GPIO_O
151P   LVDS25_4mA_SLEW-OFF_P_O   LVDS25_4mA_SLEW-OFF_GPIO_O
152N   LVDS25_4mA_SLEW-OFF_ODT-100_N_O   LVDS25_4mA_SLEW-OFF_GPIO_O
152P   LVDS25_4mA_SLEW-OFF_ODT-100_P_O   LVDS25_4mA_SLEW-OFF_GPIO_O
153N   LVDS25_3P5mA_SLEW-OFF_N_O   LVDS25_3P5mA_SLEW-OFF_GPIO_O
153P   LVDS25_3P5mA_SLEW-OFF_P_O   LVDS25_3P5mA_SLEW-OFF_GPIO_O
154N   LVDS25_3P5mA_SLEW-OFF_ODT-100_N_O   LVDS25_3P5mA_SLEW-OFF_GPIO_O
154P   LVDS25_3P5mA_SLEW-OFF_ODT-100_P_O   LVDS25_3P5mA_SLEW-OFF_GPIO_O
155N   LVDS25_3mA_SLEW-OFF_N_O   LVDS25_3mA_SLEW-OFF_GPIO_O
155P   LVDS25_3mA_SLEW-OFF_P_O   LVDS25_3mA_SLEW-OFF_GPIO_O
156N   LVDS25_3mA_SLEW-OFF_ODT-100_N_O   LVDS25_3mA_SLEW-OFF_GPIO_O
156P   LVDS25_3mA_SLEW-OFF_ODT-100_P_O   LVDS25_3mA_SLEW-OFF_GPIO_O
157N   RSDS33_4mA_SLEW-OFF_N_O   RSDS33_4mA_SLEW-OFF_GPIO_O
157P   RSDS33_4mA_SLEW-OFF_P_O   RSDS33_4mA_SLEW-OFF_GPIO_O
158N   RSDS33_4mA_SLEW-OFF_ODT-100_N_O   RSDS33_4mA_SLEW-OFF_GPIO_O
158P   RSDS33_4mA_SLEW-OFF_ODT-100_P_O   RSDS33_4mA_SLEW-OFF_GPIO_O
159N   RSDS33_3mA_SLEW-OFF_N_O   RSDS33_3mA_SLEW-OFF_GPIO_O
159P   RSDS33_3mA_SLEW-OFF_P_O   RSDS33_3mA_SLEW-OFF_GPIO_O
160N   RSDS33_3mA_SLEW-OFF_ODT-100_N_O   RSDS33_3mA_SLEW-OFF_GPIO_O
160P   RSDS33_3mA_SLEW-OFF_ODT-100_P_O   RSDS33_3mA_SLEW-OFF_GPIO_O
161N   RSDS33_2mA_SLEW-OFF_N_O   RSDS33_2mA_SLEW-OFF_GPIO_O
161P   RSDS33_2mA_SLEW-OFF_P_O   RSDS33_2mA_SLEW-OFF_GPIO_O
162N   RSDS33_2mA_SLEW-OFF_ODT-100_N_O   RSDS33_2mA_SLEW-OFF_GPIO_O
162P   RSDS33_2mA_SLEW-OFF_ODT-100_P_O   RSDS33_2mA_SLEW-OFF_GPIO_O
163N   RSDS33_1P5mA_SLEW-OFF_N_O   RSDS33_1P5mA_SLEW-OFF_GPIO_O
163P   RSDS33_1P5mA_SLEW-OFF_P_O   RSDS33_1P5mA_SLEW-OFF_GPIO_O
164N   RSDS33_1P5mA_SLEW-OFF_ODT-100_N_O   RSDS33_1P5mA_SLEW-OFF_GPIO_O
164P   RSDS33_1P5mA_SLEW-OFF_ODT-100_P_O   RSDS33_1P5mA_SLEW-OFF_GPIO_O
165N   RSDS25_4mA_SLEW-OFF_N_O   RSDS25_4mA_SLEW-OFF_GPIO_O
165P   RSDS25_4mA_SLEW-OFF_P_O   RSDS25_4mA_SLEW-OFF_GPIO_O
166N   RSDS25_4mA_SLEW-OFF_ODT-100_N_O   RSDS25_4mA_SLEW-OFF_GPIO_O
166P   RSDS25_4mA_SLEW-OFF_ODT-100_P_O   RSDS25_4mA_SLEW-OFF_GPIO_O
167N   RSDS25_3mA_SLEW-OFF_N_O   RSDS25_3mA_SLEW-OFF_GPIO_O
167P   RSDS25_3mA_SLEW-OFF_P_O   RSDS25_3mA_SLEW-OFF_GPIO_O
168N   RSDS25_3mA_SLEW-OFF_ODT-100_N_O   RSDS25_3mA_SLEW-OFF_GPIO_O
168P   RSDS25_3mA_SLEW-OFF_ODT-100_P_O   RSDS25_3mA_SLEW-OFF_GPIO_O
169N   RSDS25_2mA_SLEW-OFF_N_O   RSDS25_2mA_SLEW-OFF_GPIO_O
169P   RSDS25_2mA_SLEW-OFF_P_O   RSDS25_2mA_SLEW-OFF_GPIO_O
170N   RSDS25_2mA_SLEW-OFF_ODT-100_N_O   RSDS25_2mA_SLEW-OFF_GPIO_O
170P   RSDS25_2mA_SLEW-OFF_ODT-100_P_O   RSDS25_2mA_SLEW-OFF_GPIO_O
171N   RSDS25_1P5mA_SLEW-OFF_N_O   RSDS25_1P5mA_SLEW-OFF_GPIO_O
171P   RSDS25_1P5mA_SLEW-OFF_P_O   RSDS25_1P5mA_SLEW-OFF_GPIO_O
172N   RSDS25_1P5mA_SLEW-OFF_ODT-100_N_O   RSDS25_1P5mA_SLEW-OFF_GPIO_O
172P   RSDS25_1P5mA_SLEW-OFF_ODT-100_P_O   RSDS25_1P5mA_SLEW-OFF_GPIO_O
173N   MINILVDS33_6mA_SLEW-OFF_N_O   MINILVDS33_6mA_SLEW-OFF_GPIO_O
173P   MINILVDS33_6mA_SLEW-OFF_P_O   MINILVDS33_6mA_SLEW-OFF_GPIO_O
174N   MINILVDS33_6mA_SLEW-OFF_ODT-100_N_O   MINILVDS33_6mA_SLEW-OFF_GPIO_O
174P   MINILVDS33_6mA_SLEW-OFF_ODT-100_P_O   MINILVDS33_6mA_SLEW-OFF_GPIO_O
175N   MINILVDS33_4mA_SLEW-OFF_N_O   MINILVDS33_4mA_SLEW-OFF_GPIO_O
175P   MINILVDS33_4mA_SLEW-OFF_P_O   MINILVDS33_4mA_SLEW-OFF_GPIO_O
176N   MINILVDS33_4mA_SLEW-OFF_ODT-100_N_O   MINILVDS33_4mA_SLEW-OFF_GPIO_O
176P   MINILVDS33_4mA_SLEW-OFF_ODT-100_P_O   MINILVDS33_4mA_SLEW-OFF_GPIO_O
177N   MINILVDS33_3P5mA_SLEW-OFF_N_O   MINILVDS33_3P5mA_SLEW-OFF_GPIO_O
177P   MINILVDS33_3P5mA_SLEW-OFF_P_O   MINILVDS33_3P5mA_SLEW-OFF_GPIO_O
178N   MINILVDS33_3P5mA_SLEW-OFF_ODT-100_N_O   MINILVDS33_3P5mA_SLEW-OFF_GPIO_O
178P   MINILVDS33_3P5mA_SLEW-OFF_ODT-100_P_O   MINILVDS33_3P5mA_SLEW-OFF_GPIO_O
179N   MINILVDS33_3mA_SLEW-OFF_N_O   MINILVDS33_3mA_SLEW-OFF_GPIO_O
179P   MINILVDS33_3mA_SLEW-OFF_P_O   MINILVDS33_3mA_SLEW-OFF_GPIO_O
180N   MINILVDS33_3mA_SLEW-OFF_ODT-100_N_O   MINILVDS33_3mA_SLEW-OFF_GPIO_O
180P   MINILVDS33_3mA_SLEW-OFF_ODT-100_P_O   MINILVDS33_3mA_SLEW-OFF_GPIO_O
181N   MINILVDS25_6mA_SLEW-OFF_N_O   MINILVDS25_6mA_SLEW-OFF_GPIO_O
181P   MINILVDS25_6mA_SLEW-OFF_P_O   MINILVDS25_6mA_SLEW-OFF_GPIO_O
182N   MINILVDS25_6mA_SLEW-OFF_ODT-100_N_O   MINILVDS25_6mA_SLEW-OFF_GPIO_O
182P   MINILVDS25_6mA_SLEW-OFF_ODT-100_P_O   MINILVDS25_6mA_SLEW-OFF_GPIO_O
183N   MINILVDS25_4mA_SLEW-OFF_N_O   MINILVDS25_4mA_SLEW-OFF_GPIO_O
183P   MINILVDS25_4mA_SLEW-OFF_P_O   MINILVDS25_4mA_SLEW-OFF_GPIO_O
184N   MINILVDS25_4mA_SLEW-OFF_ODT-100_N_O   MINILVDS25_4mA_SLEW-OFF_GPIO_O
184P   MINILVDS25_4mA_SLEW-OFF_ODT-100_P_O   MINILVDS25_4mA_SLEW-OFF_GPIO_O
185N   MINILVDS25_3P5mA_SLEW-OFF_N_O   MINILVDS25_3P5mA_SLEW-OFF_GPIO_O
185P   MINILVDS25_3P5mA_SLEW-OFF_P_O   MINILVDS25_3P5mA_SLEW-OFF_GPIO_O
186N   MINILVDS25_3P5mA_SLEW-OFF_ODT-100_N_O   MINILVDS25_3P5mA_SLEW-OFF_GPIO_O
186P   MINILVDS25_3P5mA_SLEW-OFF_ODT-100_P_O   MINILVDS25_3P5mA_SLEW-OFF_GPIO_O
187N   MINILVDS25_3mA_SLEW-OFF_N_O   MINILVDS25_3mA_SLEW-OFF_GPIO_O
187P   MINILVDS25_3mA_SLEW-OFF_P_O   MINILVDS25_3mA_SLEW-OFF_GPIO_O
188N   MINILVDS25_3mA_SLEW-OFF_ODT-100_N_O   MINILVDS25_3mA_SLEW-OFF_GPIO_O
188P   MINILVDS25_3mA_SLEW-OFF_ODT-100_P_O   MINILVDS25_3mA_SLEW-OFF_GPIO_O
189N   SUBLVDS33_3mA_SLEW-OFF_N_O   SUBLVDS33_3mA_SLEW-OFF_GPIO_O
189P   SUBLVDS33_3mA_SLEW-OFF_P_O   SUBLVDS33_3mA_SLEW-OFF_GPIO_O
190N   SUBLVDS33_3mA_SLEW-OFF_ODT-100_N_O   SUBLVDS33_3mA_SLEW-OFF_GPIO_O
190P   SUBLVDS33_3mA_SLEW-OFF_ODT-100_P_O   SUBLVDS33_3mA_SLEW-OFF_GPIO_O
191N   SUBLVDS33_2mA_SLEW-OFF_N_O   SUBLVDS33_2mA_SLEW-OFF_GPIO_O
191P   SUBLVDS33_2mA_SLEW-OFF_P_O   SUBLVDS33_2mA_SLEW-OFF_GPIO_O
192N   SUBLVDS33_2mA_SLEW-OFF_ODT-100_N_O   SUBLVDS33_2mA_SLEW-OFF_GPIO_O
192P   SUBLVDS33_2mA_SLEW-OFF_ODT-100_P_O   SUBLVDS33_2mA_SLEW-OFF_GPIO_O
193N   SUBLVDS33_1P5mA_SLEW-OFF_N_O   SUBLVDS33_1P5mA_SLEW-OFF_GPIO_O
193P   SUBLVDS33_1P5mA_SLEW-OFF_P_O   SUBLVDS33_1P5mA_SLEW-OFF_GPIO_O
194N   SUBLVDS33_1P5mA_SLEW-OFF_ODT-100_N_O   SUBLVDS33_1P5mA_SLEW-OFF_GPIO_O
194P   SUBLVDS33_1P5mA_SLEW-OFF_ODT-100_P_O   SUBLVDS33_1P5mA_SLEW-OFF_GPIO_O
195N   SUBLVDS33_1mA_SLEW-OFF_N_O   SUBLVDS33_1mA_SLEW-OFF_GPIO_O
195P   SUBLVDS33_1mA_SLEW-OFF_P_O   SUBLVDS33_1mA_SLEW-OFF_GPIO_O
196N   SUBLVDS33_1mA_SLEW-OFF_ODT-100_N_O   SUBLVDS33_1mA_SLEW-OFF_GPIO_O
196P   SUBLVDS33_1mA_SLEW-OFF_ODT-100_P_O   SUBLVDS33_1mA_SLEW-OFF_GPIO_O
197N   SUBLVDS25_3mA_SLEW-OFF_N_O   SUBLVDS25_3mA_SLEW-OFF_GPIO_O
197P   SUBLVDS25_3mA_SLEW-OFF_P_O   SUBLVDS25_3mA_SLEW-OFF_GPIO_O
198N   SUBLVDS25_3mA_SLEW-OFF_ODT-100_N_O   SUBLVDS25_3mA_SLEW-OFF_GPIO_O
198P   SUBLVDS25_3mA_SLEW-OFF_ODT-100_P_O   SUBLVDS25_3mA_SLEW-OFF_GPIO_O
199N   SUBLVDS25_2mA_SLEW-OFF_N_O   SUBLVDS25_2mA_SLEW-OFF_GPIO_O
199P   SUBLVDS25_2mA_SLEW-OFF_P_O   SUBLVDS25_2mA_SLEW-OFF_GPIO_O
200N   SUBLVDS25_2mA_SLEW-OFF_ODT-100_N_O   SUBLVDS25_2mA_SLEW-OFF_GPIO_O
200P   SUBLVDS25_2mA_SLEW-OFF_ODT-100_P_O   SUBLVDS25_2mA_SLEW-OFF_GPIO_O
201N   SUBLVDS25_1P5mA_SLEW-OFF_N_O   SUBLVDS25_1P5mA_SLEW-OFF_GPIO_O
201P   SUBLVDS25_1P5mA_SLEW-OFF_P_O   SUBLVDS25_1P5mA_SLEW-OFF_GPIO_O
202N   SUBLVDS25_1P5mA_SLEW-OFF_ODT-100_N_O   SUBLVDS25_1P5mA_SLEW-OFF_GPIO_O
202P   SUBLVDS25_1P5mA_SLEW-OFF_ODT-100_P_O   SUBLVDS25_1P5mA_SLEW-OFF_GPIO_O
203N   SUBLVDS25_1mA_SLEW-OFF_N_O   SUBLVDS25_1mA_SLEW-OFF_GPIO_O
203P   SUBLVDS25_1mA_SLEW-OFF_P_O   SUBLVDS25_1mA_SLEW-OFF_GPIO_O
204N   SUBLVDS25_1mA_SLEW-OFF_ODT-100_N_O   SUBLVDS25_1mA_SLEW-OFF_GPIO_O
204P   SUBLVDS25_1mA_SLEW-OFF_ODT-100_P_O   SUBLVDS25_1mA_SLEW-OFF_GPIO_O
205N   PPDS33_4mA_SLEW-OFF_N_O   PPDS33_4mA_SLEW-OFF_GPIO_O
205P   PPDS33_4mA_SLEW-OFF_P_O   PPDS33_4mA_SLEW-OFF_GPIO_O
206N   PPDS33_4mA_SLEW-OFF_ODT-100_N_O   PPDS33_4mA_SLEW-OFF_GPIO_O
206P   PPDS33_4mA_SLEW-OFF_ODT-100_P_O   PPDS33_4mA_SLEW-OFF_GPIO_O
207N   PPDS33_3mA_SLEW-OFF_N_O   PPDS33_3mA_SLEW-OFF_GPIO_O
207P   PPDS33_3mA_SLEW-OFF_P_O   PPDS33_3mA_SLEW-OFF_GPIO_O
208N   PPDS33_3mA_SLEW-OFF_ODT-100_N_O   PPDS33_3mA_SLEW-OFF_GPIO_O
208P   PPDS33_3mA_SLEW-OFF_ODT-100_P_O   PPDS33_3mA_SLEW-OFF_GPIO_O
209N   PPDS33_2mA_SLEW-OFF_N_O   PPDS33_2mA_SLEW-OFF_GPIO_O
209P   PPDS33_2mA_SLEW-OFF_P_O   PPDS33_2mA_SLEW-OFF_GPIO_O
210N   PPDS33_2mA_SLEW-OFF_ODT-100_N_O   PPDS33_2mA_SLEW-OFF_GPIO_O
210P   PPDS33_2mA_SLEW-OFF_ODT-100_P_O   PPDS33_2mA_SLEW-OFF_GPIO_O
211N   PPDS33_1P5mA_SLEW-OFF_N_O   PPDS33_1P5mA_SLEW-OFF_GPIO_O
211P   PPDS33_1P5mA_SLEW-OFF_P_O   PPDS33_1P5mA_SLEW-OFF_GPIO_O
212N   PPDS33_1P5mA_SLEW-OFF_ODT-100_N_O   PPDS33_1P5mA_SLEW-OFF_GPIO_O
212P   PPDS33_1P5mA_SLEW-OFF_ODT-100_P_O   PPDS33_1P5mA_SLEW-OFF_GPIO_O
213N   PPDS25_4mA_SLEW-OFF_N_O   PPDS25_4mA_SLEW-OFF_GPIO_O
213P   PPDS25_4mA_SLEW-OFF_P_O   PPDS25_4mA_SLEW-OFF_GPIO_O
214N   PPDS25_4mA_SLEW-OFF_ODT-100_N_O   PPDS25_4mA_SLEW-OFF_GPIO_O
214P   PPDS25_4mA_SLEW-OFF_ODT-100_P_O   PPDS25_4mA_SLEW-OFF_GPIO_O
215N   PPDS25_3mA_SLEW-OFF_N_O   PPDS25_3mA_SLEW-OFF_GPIO_O
215P   PPDS25_3mA_SLEW-OFF_P_O   PPDS25_3mA_SLEW-OFF_GPIO_O
216N   PPDS25_3mA_SLEW-OFF_ODT-100_N_O   PPDS25_3mA_SLEW-OFF_GPIO_O
216P   PPDS25_3mA_SLEW-OFF_ODT-100_P_O   PPDS25_3mA_SLEW-OFF_GPIO_O
217N   PPDS25_2mA_SLEW-OFF_N_O   PPDS25_2mA_SLEW-OFF_GPIO_O
217P   PPDS25_2mA_SLEW-OFF_P_O   PPDS25_2mA_SLEW-OFF_GPIO_O
218N   PPDS25_2mA_SLEW-OFF_ODT-100_N_O   PPDS25_2mA_SLEW-OFF_GPIO_O
218P   PPDS25_2mA_SLEW-OFF_ODT-100_P_O   PPDS25_2mA_SLEW-OFF_GPIO_O
219N   PPDS25_1P5mA_SLEW-OFF_N_O   PPDS25_1P5mA_SLEW-OFF_GPIO_O
219P   PPDS25_1P5mA_SLEW-OFF_P_O   PPDS25_1P5mA_SLEW-OFF_GPIO_O
220N   PPDS25_1P5mA_SLEW-OFF_ODT-100_N_O   PPDS25_1P5mA_SLEW-OFF_GPIO_O
220P   PPDS25_1P5mA_SLEW-OFF_ODT-100_P_O   PPDS25_1P5mA_SLEW-OFF_GPIO_O
221N   LCMDS33_6mA_SLEW-OFF_N_O   LCMDS33_6mA_SLEW-OFF_GPIO_O
221P   LCMDS33_6mA_SLEW-OFF_P_O   LCMDS33_6mA_SLEW-OFF_GPIO_O
222N   LCMDS33_6mA_SLEW-OFF_ODT-100_N_O   LCMDS33_6mA_SLEW-OFF_GPIO_O
222P   LCMDS33_6mA_SLEW-OFF_ODT-100_P_O   LCMDS33_6mA_SLEW-OFF_GPIO_O
223N   LCMDS33_4mA_SLEW-OFF_N_O   LCMDS33_4mA_SLEW-OFF_GPIO_O
223P   LCMDS33_4mA_SLEW-OFF_P_O   LCMDS33_4mA_SLEW-OFF_GPIO_O
224N   LCMDS33_4mA_SLEW-OFF_ODT-100_N_O   LCMDS33_4mA_SLEW-OFF_GPIO_O
224P   LCMDS33_4mA_SLEW-OFF_ODT-100_P_O   LCMDS33_4mA_SLEW-OFF_GPIO_O
225N   LCMDS33_3P5mA_SLEW-OFF_N_O   LCMDS33_3P5mA_SLEW-OFF_GPIO_O
225P   LCMDS33_3P5mA_SLEW-OFF_P_O   LCMDS33_3P5mA_SLEW-OFF_GPIO_O
226N   LCMDS33_3P5mA_SLEW-OFF_ODT-100_N_O   LCMDS33_3P5mA_SLEW-OFF_GPIO_O
226P   LCMDS33_3P5mA_SLEW-OFF_ODT-100_P_O   LCMDS33_3P5mA_SLEW-OFF_GPIO_O
227N   LCMDS33_3mA_SLEW-OFF_N_O   LCMDS33_3mA_SLEW-OFF_GPIO_O
227P   LCMDS33_3mA_SLEW-OFF_P_O   LCMDS33_3mA_SLEW-OFF_GPIO_O
228N   LCMDS33_3mA_SLEW-OFF_ODT-100_N_O   LCMDS33_3mA_SLEW-OFF_GPIO_O
228P   LCMDS33_3mA_SLEW-OFF_ODT-100_P_O   LCMDS33_3mA_SLEW-OFF_GPIO_O
229N   LCMDS25_6mA_SLEW-OFF_N_O   LCMDS25_6mA_SLEW-OFF_GPIO_O
229P   LCMDS25_6mA_SLEW-OFF_P_O   LCMDS25_6mA_SLEW-OFF_GPIO_O
230N   LCMDS25_6mA_SLEW-OFF_ODT-100_N_O   LCMDS25_6mA_SLEW-OFF_GPIO_O
230P   LCMDS25_6mA_SLEW-OFF_ODT-100_P_O   LCMDS25_6mA_SLEW-OFF_GPIO_O
231N   LCMDS25_4mA_SLEW-OFF_N_O   LCMDS25_4mA_SLEW-OFF_GPIO_O
231P   LCMDS25_4mA_SLEW-OFF_P_O   LCMDS25_4mA_SLEW-OFF_GPIO_O
232N   LCMDS25_4mA_SLEW-OFF_ODT-100_N_O   LCMDS25_4mA_SLEW-OFF_GPIO_O
232P   LCMDS25_4mA_SLEW-OFF_ODT-100_P_O   LCMDS25_4mA_SLEW-OFF_GPIO_O
233N   LCMDS25_3P5mA_SLEW-OFF_N_O   LCMDS25_3P5mA_SLEW-OFF_GPIO_O
233P   LCMDS25_3P5mA_SLEW-OFF_P_O   LCMDS25_3P5mA_SLEW-OFF_GPIO_O
234N   LCMDS25_3P5mA_SLEW-OFF_ODT-100_N_O   LCMDS25_3P5mA_SLEW-OFF_GPIO_O
234P   LCMDS25_3P5mA_SLEW-OFF_ODT-100_P_O   LCMDS25_3P5mA_SLEW-OFF_GPIO_O
235N   LCMDS25_3mA_SLEW-OFF_N_O   LCMDS25_3mA_SLEW-OFF_GPIO_O
235P   LCMDS25_3mA_SLEW-OFF_P_O   LCMDS25_3mA_SLEW-OFF_GPIO_O
236N   LCMDS25_3mA_SLEW-OFF_ODT-100_N_O   LCMDS25_3mA_SLEW-OFF_GPIO_O
236P   LCMDS25_3mA_SLEW-OFF_ODT-100_P_O   LCMDS25_3mA_SLEW-OFF_GPIO_O
237N   LVDS33_CL_ODT-OFF_HYST-OFF_N_I   LVDS33_CL_ODT-OFF_HYST-OFF_GPIO_I
237P   LVDS33_CL_ODT-OFF_HYST-OFF_P_I   LVDS33_CL_ODT-OFF_HYST-OFF_GPIO_I
238N   LVDS33_CL_ODT-100_HYST-OFF_N_I   LVDS33_CL_ODT-OFF_HYST-OFF_GPIO_I
238P   LVDS33_CL_ODT-100_HYST-OFF_P_I   LVDS33_CL_ODT-OFF_HYST-OFF_GPIO_I
239N   LVDS25_CL_ODT-OFF_HYST-OFF_N_I   LVDS25_CL_ODT-OFF_HYST-OFF_GPIO_I
239P   LVDS25_CL_ODT-OFF_HYST-OFF_P_I   LVDS25_CL_ODT-OFF_HYST-OFF_GPIO_I
240N   LVDS25_CL_ODT-100_HYST-OFF_N_I   LVDS25_CL_ODT-OFF_HYST-OFF_GPIO_I
240P   LVDS25_CL_ODT-100_HYST-OFF_P_I   LVDS25_CL_ODT-OFF_HYST-OFF_GPIO_I
241N   LVDS25_18_ODT-OFF_HYST-OFF_N_I   LVDS25_18_ODT-OFF_HYST-OFF_GPIO_I
241P   LVDS25_18_ODT-OFF_HYST-OFF_P_I   LVDS25_18_ODT-OFF_HYST-OFF_GPIO_I
242N   LVDS25_18_ODT-100_HYST-OFF_N_I   LVDS25_18_ODT-OFF_HYST-OFF_GPIO_I
242P   LVDS25_18_ODT-100_HYST-OFF_P_I   LVDS25_18_ODT-OFF_HYST-OFF_GPIO_I
243N   LVDS25_15_ODT-OFF_HYST-OFF_N_I   LVDS25_15_ODT-OFF_HYST-OFF_GPIO_I
243P   LVDS25_15_ODT-OFF_HYST-OFF_P_I   LVDS25_15_ODT-OFF_HYST-OFF_GPIO_I
244N   LVDS25_15_ODT-100_HYST-OFF_N_I   LVDS25_15_ODT-OFF_HYST-OFF_GPIO_I
244P   LVDS25_15_ODT-100_HYST-OFF_P_I   LVDS25_15_ODT-OFF_HYST-OFF_GPIO_I
245N   LVDS25_12_ODT-OFF_HYST-OFF_N_I   LVDS25_12_ODT-OFF_HYST-OFF_GPIO_I
245P   LVDS25_12_ODT-OFF_HYST-OFF_P_I   LVDS25_12_ODT-OFF_HYST-OFF_GPIO_I
246N   LVDS25_12_ODT-100_HYST-OFF_N_I   LVDS25_12_ODT-OFF_HYST-OFF_GPIO_I
246P   LVDS25_12_ODT-100_HYST-OFF_P_I   LVDS25_12_ODT-OFF_HYST-OFF_GPIO_I
247N   RSDS33_CL_ODT-OFF_HYST-OFF_N_I   RSDS33_CL_ODT-OFF_HYST-OFF_GPIO_I
247P   RSDS33_CL_ODT-OFF_HYST-OFF_P_I   RSDS33_CL_ODT-OFF_HYST-OFF_GPIO_I
248N   RSDS33_CL_ODT-100_HYST-OFF_N_I   RSDS33_CL_ODT-OFF_HYST-OFF_GPIO_I
248P   RSDS33_CL_ODT-100_HYST-OFF_P_I   RSDS33_CL_ODT-OFF_HYST-OFF_GPIO_I
249N   RSDS25_CL_ODT-OFF_HYST-OFF_N_I   RSDS25_CL_ODT-OFF_HYST-OFF_GPIO_I
249P   RSDS25_CL_ODT-OFF_HYST-OFF_P_I   RSDS25_CL_ODT-OFF_HYST-OFF_GPIO_I
250N   RSDS25_CL_ODT-100_HYST-OFF_N_I   RSDS25_CL_ODT-OFF_HYST-OFF_GPIO_I
250P   RSDS25_CL_ODT-100_HYST-OFF_P_I   RSDS25_CL_ODT-OFF_HYST-OFF_GPIO_I
251N   RSDS25_18_ODT-OFF_HYST-OFF_N_I   RSDS25_18_ODT-OFF_HYST-OFF_GPIO_I
251P   RSDS25_18_ODT-OFF_HYST-OFF_P_I   RSDS25_18_ODT-OFF_HYST-OFF_GPIO_I
252N   RSDS25_18_ODT-100_HYST-OFF_N_I   RSDS25_18_ODT-OFF_HYST-OFF_GPIO_I
252P   RSDS25_18_ODT-100_HYST-OFF_P_I   RSDS25_18_ODT-OFF_HYST-OFF_GPIO_I
253N   RSDS25_15_ODT-OFF_HYST-OFF_N_I   RSDS25_15_ODT-OFF_HYST-OFF_GPIO_I
253P   RSDS25_15_ODT-OFF_HYST-OFF_P_I   RSDS25_15_ODT-OFF_HYST-OFF_GPIO_I
254N   RSDS25_15_ODT-100_HYST-OFF_N_I   RSDS25_15_ODT-OFF_HYST-OFF_GPIO_I
254P   RSDS25_15_ODT-100_HYST-OFF_P_I   RSDS25_15_ODT-OFF_HYST-OFF_GPIO_I
255N   RSDS25_12_ODT-OFF_HYST-OFF_N_I   RSDS25_12_ODT-OFF_HYST-OFF_GPIO_I
255P   RSDS25_12_ODT-OFF_HYST-OFF_P_I   RSDS25_12_ODT-OFF_HYST-OFF_GPIO_I
256N   RSDS25_12_ODT-100_HYST-OFF_N_I   RSDS25_12_ODT-OFF_HYST-OFF_GPIO_I
256P   RSDS25_12_ODT-100_HYST-OFF_P_I   RSDS25_12_ODT-OFF_HYST-OFF_GPIO_I
257N   MINILVDS33_CL_ODT-OFF_HYST-OFF_N_I   MINILVDS33_CL_ODT-OFF_HYST-OFF_GPIO_I
257P   MINILVDS33_CL_ODT-OFF_HYST-OFF_P_I   MINILVDS33_CL_ODT-OFF_HYST-OFF_GPIO_I
258N   MINILVDS33_CL_ODT-100_HYST-OFF_N_I   MINILVDS33_CL_ODT-OFF_HYST-OFF_GPIO_I
258P   MINILVDS33_CL_ODT-100_HYST-OFF_P_I   MINILVDS33_CL_ODT-OFF_HYST-OFF_GPIO_I
259N   MINILVDS25_CL_ODT-OFF_HYST-OFF_N_I   MINILVDS25_CL_ODT-OFF_HYST-OFF_GPIO_I
259P   MINILVDS25_CL_ODT-OFF_HYST-OFF_P_I   MINILVDS25_CL_ODT-OFF_HYST-OFF_GPIO_I
260N   MINILVDS25_CL_ODT-100_HYST-OFF_N_I   MINILVDS25_CL_ODT-OFF_HYST-OFF_GPIO_I
260P   MINILVDS25_CL_ODT-100_HYST-OFF_P_I   MINILVDS25_CL_ODT-OFF_HYST-OFF_GPIO_I
261N   MINILVDS25_18_ODT-OFF_HYST-OFF_N_I   MINILVDS25_18_ODT-OFF_HYST-OFF_GPIO_I
261P   MINILVDS25_18_ODT-OFF_HYST-OFF_P_I   MINILVDS25_18_ODT-OFF_HYST-OFF_GPIO_I
262N   MINILVDS25_18_ODT-100_HYST-OFF_N_I   MINILVDS25_18_ODT-OFF_HYST-OFF_GPIO_I
262P   MINILVDS25_18_ODT-100_HYST-OFF_P_I   MINILVDS25_18_ODT-OFF_HYST-OFF_GPIO_I
263N   MINILVDS25_15_ODT-OFF_HYST-OFF_N_I   MINILVDS25_15_ODT-OFF_HYST-OFF_GPIO_I
263P   MINILVDS25_15_ODT-OFF_HYST-OFF_P_I   MINILVDS25_15_ODT-OFF_HYST-OFF_GPIO_I
264N   MINILVDS25_15_ODT-100_HYST-OFF_N_I   MINILVDS25_15_ODT-OFF_HYST-OFF_GPIO_I
264P   MINILVDS25_15_ODT-100_HYST-OFF_P_I   MINILVDS25_15_ODT-OFF_HYST-OFF_GPIO_I
265N   MINILVDS25_12_ODT-OFF_HYST-OFF_N_I   MINILVDS25_12_ODT-OFF_HYST-OFF_GPIO_I
265P   MINILVDS25_12_ODT-OFF_HYST-OFF_P_I   MINILVDS25_12_ODT-OFF_HYST-OFF_GPIO_I
266N   MINILVDS25_12_ODT-100_HYST-OFF_N_I   MINILVDS25_12_ODT-OFF_HYST-OFF_GPIO_I
266P   MINILVDS25_12_ODT-100_HYST-OFF_P_I   MINILVDS25_12_ODT-OFF_HYST-OFF_GPIO_I
267N   SUBLVDS33_CL_ODT-OFF_HYST-OFF_N_I   SUBLVDS33_CL_ODT-OFF_HYST-OFF_GPIO_I
267P   SUBLVDS33_CL_ODT-OFF_HYST-OFF_P_I   SUBLVDS33_CL_ODT-OFF_HYST-OFF_GPIO_I
268N   SUBLVDS33_CL_ODT-100_HYST-OFF_N_I   SUBLVDS33_CL_ODT-OFF_HYST-OFF_GPIO_I
268P   SUBLVDS33_CL_ODT-100_HYST-OFF_P_I   SUBLVDS33_CL_ODT-OFF_HYST-OFF_GPIO_I
269N   SUBLVDS25_CL_ODT-OFF_HYST-OFF_N_I   SUBLVDS25_CL_ODT-OFF_HYST-OFF_GPIO_I
269P   SUBLVDS25_CL_ODT-OFF_HYST-OFF_P_I   SUBLVDS25_CL_ODT-OFF_HYST-OFF_GPIO_I
270N   SUBLVDS25_CL_ODT-100_HYST-OFF_N_I   SUBLVDS25_CL_ODT-OFF_HYST-OFF_GPIO_I
270P   SUBLVDS25_CL_ODT-100_HYST-OFF_P_I   SUBLVDS25_CL_ODT-OFF_HYST-OFF_GPIO_I
271N   SUBLVDS25_18_ODT-OFF_HYST-OFF_N_I   SUBLVDS25_18_ODT-OFF_HYST-OFF_GPIO_I
271P   SUBLVDS25_18_ODT-OFF_HYST-OFF_P_I   SUBLVDS25_18_ODT-OFF_HYST-OFF_GPIO_I
272N   SUBLVDS25_18_ODT-100_HYST-OFF_N_I   SUBLVDS25_18_ODT-OFF_HYST-OFF_GPIO_I
272P   SUBLVDS25_18_ODT-100_HYST-OFF_P_I   SUBLVDS25_18_ODT-OFF_HYST-OFF_GPIO_I
273N   SUBLVDS25_15_ODT-OFF_HYST-OFF_N_I   SUBLVDS25_15_ODT-OFF_HYST-OFF_GPIO_I
273P   SUBLVDS25_15_ODT-OFF_HYST-OFF_P_I   SUBLVDS25_15_ODT-OFF_HYST-OFF_GPIO_I
274N   SUBLVDS25_15_ODT-100_HYST-OFF_N_I   SUBLVDS25_15_ODT-OFF_HYST-OFF_GPIO_I
274P   SUBLVDS25_15_ODT-100_HYST-OFF_P_I   SUBLVDS25_15_ODT-OFF_HYST-OFF_GPIO_I
275N   SUBLVDS25_12_ODT-OFF_HYST-OFF_N_I   SUBLVDS25_12_ODT-OFF_HYST-OFF_GPIO_I
275P   SUBLVDS25_12_ODT-OFF_HYST-OFF_P_I   SUBLVDS25_12_ODT-OFF_HYST-OFF_GPIO_I
276N   SUBLVDS25_12_ODT-100_HYST-OFF_N_I   SUBLVDS25_12_ODT-OFF_HYST-OFF_GPIO_I
276P   SUBLVDS25_12_ODT-100_HYST-OFF_P_I   SUBLVDS25_12_ODT-OFF_HYST-OFF_GPIO_I
277N   PPDS33_CL_ODT-OFF_HYST-OFF_N_I   PPDS33_CL_ODT-OFF_HYST-OFF_GPIO_I
277P   PPDS33_CL_ODT-OFF_HYST-OFF_P_I   PPDS33_CL_ODT-OFF_HYST-OFF_GPIO_I
278N   PPDS33_CL_ODT-100_HYST-OFF_N_I   PPDS33_CL_ODT-OFF_HYST-OFF_GPIO_I
278P   PPDS33_CL_ODT-100_HYST-OFF_P_I   PPDS33_CL_ODT-OFF_HYST-OFF_GPIO_I
279N   PPDS25_CL_ODT-OFF_HYST-OFF_N_I   PPDS25_CL_ODT-OFF_HYST-OFF_GPIO_I
279P   PPDS25_CL_ODT-OFF_HYST-OFF_P_I   PPDS25_CL_ODT-OFF_HYST-OFF_GPIO_I
280N   PPDS25_CL_ODT-100_HYST-OFF_N_I   PPDS25_CL_ODT-OFF_HYST-OFF_GPIO_I
280P   PPDS25_CL_ODT-100_HYST-OFF_P_I   PPDS25_CL_ODT-OFF_HYST-OFF_GPIO_I
281N   PPDS25_18_ODT-OFF_HYST-OFF_N_I   PPDS25_18_ODT-OFF_HYST-OFF_GPIO_I
281P   PPDS25_18_ODT-OFF_HYST-OFF_P_I   PPDS25_18_ODT-OFF_HYST-OFF_GPIO_I
282N   PPDS25_18_ODT-100_HYST-OFF_N_I   PPDS25_18_ODT-OFF_HYST-OFF_GPIO_I
282P   PPDS25_18_ODT-100_HYST-OFF_P_I   PPDS25_18_ODT-OFF_HYST-OFF_GPIO_I
283N   PPDS25_15_ODT-OFF_HYST-OFF_N_I   PPDS25_15_ODT-OFF_HYST-OFF_GPIO_I
283P   PPDS25_15_ODT-OFF_HYST-OFF_P_I   PPDS25_15_ODT-OFF_HYST-OFF_GPIO_I
284N   PPDS25_15_ODT-100_HYST-OFF_N_I   PPDS25_15_ODT-OFF_HYST-OFF_GPIO_I
284P   PPDS25_15_ODT-100_HYST-OFF_P_I   PPDS25_15_ODT-OFF_HYST-OFF_GPIO_I
285N   PPDS25_12_ODT-OFF_HYST-OFF_N_I   PPDS25_12_ODT-OFF_HYST-OFF_GPIO_I
285P   PPDS25_12_ODT-OFF_HYST-OFF_P_I   PPDS25_12_ODT-OFF_HYST-OFF_GPIO_I
286N   PPDS25_12_ODT-100_HYST-OFF_N_I   PPDS25_12_ODT-OFF_HYST-OFF_GPIO_I
286P   PPDS25_12_ODT-100_HYST-OFF_P_I   PPDS25_12_ODT-OFF_HYST-OFF_GPIO_I
287N   LCMDS33_CL_ODT-OFF_HYST-OFF_N_I   LCMDS33_CL_ODT-OFF_HYST-OFF_GPIO_I
287P   LCMDS33_CL_ODT-OFF_HYST-OFF_P_I   LCMDS33_CL_ODT-OFF_HYST-OFF_GPIO_I
288N   LCMDS33_CL_ODT-100_HYST-OFF_N_I   LCMDS33_CL_ODT-OFF_HYST-OFF_GPIO_I
288P   LCMDS33_CL_ODT-100_HYST-OFF_P_I   LCMDS33_CL_ODT-OFF_HYST-OFF_GPIO_I
289N   LCMDS25_CL_ODT-OFF_HYST-OFF_N_I   LCMDS25_CL_ODT-OFF_HYST-OFF_GPIO_I
289P   LCMDS25_CL_ODT-OFF_HYST-OFF_P_I   LCMDS25_CL_ODT-OFF_HYST-OFF_GPIO_I
290N   LCMDS25_CL_ODT-100_HYST-OFF_N_I   LCMDS25_CL_ODT-OFF_HYST-OFF_GPIO_I
290P   LCMDS25_CL_ODT-100_HYST-OFF_P_I   LCMDS25_CL_ODT-OFF_HYST-OFF_GPIO_I
291N   LCMDS25_18_ODT-OFF_HYST-OFF_N_I   LCMDS25_18_ODT-OFF_HYST-OFF_GPIO_I
291P   LCMDS25_18_ODT-OFF_HYST-OFF_P_I   LCMDS25_18_ODT-OFF_HYST-OFF_GPIO_I
292N   LCMDS25_18_ODT-100_HYST-OFF_N_I   LCMDS25_18_ODT-OFF_HYST-OFF_GPIO_I
292P   LCMDS25_18_ODT-100_HYST-OFF_P_I   LCMDS25_18_ODT-OFF_HYST-OFF_GPIO_I
293N   LCMDS25_15_ODT-OFF_HYST-OFF_N_I   LCMDS25_15_ODT-OFF_HYST-OFF_GPIO_I
293P   LCMDS25_15_ODT-OFF_HYST-OFF_P_I   LCMDS25_15_ODT-OFF_HYST-OFF_GPIO_I
294N   LCMDS25_15_ODT-100_HYST-OFF_N_I   LCMDS25_15_ODT-OFF_HYST-OFF_GPIO_I
294P   LCMDS25_15_ODT-100_HYST-OFF_P_I   LCMDS25_15_ODT-OFF_HYST-OFF_GPIO_I
295N   LCMDS25_12_ODT-OFF_HYST-OFF_N_I   LCMDS25_12_ODT-OFF_HYST-OFF_GPIO_I
295P   LCMDS25_12_ODT-OFF_HYST-OFF_P_I   LCMDS25_12_ODT-OFF_HYST-OFF_GPIO_I
296N   LCMDS25_12_ODT-100_HYST-OFF_N_I   LCMDS25_12_ODT-OFF_HYST-OFF_GPIO_I
296P   LCMDS25_12_ODT-100_HYST-OFF_P_I   LCMDS25_12_ODT-OFF_HYST-OFF_GPIO_I
297N   HCSL33_CL_ODT-OFF_HYST-OFF_N_I   HCSL33_CL_ODT-OFF_HYST-OFF_GPIO_I
297P   HCSL33_CL_ODT-OFF_HYST-OFF_P_I   HCSL33_CL_ODT-OFF_HYST-OFF_GPIO_I
298N   HCSL33_CL_ODT-100_HYST-OFF_N_I   HCSL33_CL_ODT-OFF_HYST-OFF_GPIO_I
298P   HCSL33_CL_ODT-100_HYST-OFF_P_I   HCSL33_CL_ODT-OFF_HYST-OFF_GPIO_I
299N   HCSL25_CL_ODT-OFF_HYST-OFF_N_I   HCSL25_CL_ODT-OFF_HYST-OFF_GPIO_I
299P   HCSL25_CL_ODT-OFF_HYST-OFF_P_I   HCSL25_CL_ODT-OFF_HYST-OFF_GPIO_I
300N   HCSL25_CL_ODT-100_HYST-OFF_N_I   HCSL25_CL_ODT-OFF_HYST-OFF_GPIO_I
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[Pin Mapping]   pulldown_ref   pullup_ref   gnd_clamp_ref   power_clamp_ref   ext_ref
1N   VSS   VDDI   VSS   VDDI
1P   VSS   VDDI   VSS   VDDI
2N   VSS   VDDI   VSS   VDDI
2P   VSS   VDDI   VSS   VDDI
3N   VSS   VDDI   VSS   VDDI
3P   VSS   VDDI   VSS   VDDI
4N   VSS   VDDI   VSS   VDDI
4P   VSS   VDDI   VSS   VDDI
5N   VSS   VDDI   VSS   VDDI
5P   VSS   VDDI   VSS   VDDI
6N   VSS   VDDI   VSS   VDDI
6P   VSS   VDDI   VSS   VDDI
7N   VSS   VDDI   VSS   VDDI
7P   VSS   VDDI   VSS   VDDI
8N   VSS   VDDI   VSS   VDDI
8P   VSS   VDDI   VSS   VDDI
9N   VSS   VDDI   VSS   VDDI
9P   VSS   VDDI   VSS   VDDI
10N   VSS   VDDI   VSS   VDDI
10P   VSS   VDDI   VSS   VDDI
11N   VSS   VDDI   VSS   VDDI
11P   VSS   VDDI   VSS   VDDI
12N   VSS   VDDI   VSS   VDDI
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| Models and submodels in the file (311): LVCMOS33_8mA_SLEW-ON_GPIO_O (Output), LVCMOS33_8mA_SLEW-OFF_GPIO_O (Output), LVCMOS33_2mA_SLEW-ON_GPIO_O (Output), LVCMOS33_2mA_SLEW-OFF_GPIO_O (Output), LVCMOS33_4mA_SLEW-ON_GPIO_O (Output), LVCMOS33_4mA_SLEW-OFF_GPIO_O (Output), LVCMOS33_12mA_SLEW-ON_GPIO_O (Output), LVCMOS33_12mA_SLEW-OFF_GPIO_O (Output), LVCMOS33_16mA_SLEW-ON_GPIO_O (Output), LVCMOS33_16mA_SLEW-OFF_GPIO_O (Output), LVCMOS33_20mA_SLEW-ON_GPIO_O (Output), LVCMOS33_20mA_SLEW-OFF_GPIO_O (Output), LVCMOS25_8mA_SLEW-ON_GPIO_O (Output), LVCMOS25_8mA_SLEW-OFF_GPIO_O (Output), LVCMOS25_2mA_SLEW-ON_GPIO_O (Output), LVCMOS25_2mA_SLEW-OFF_GPIO_O (Output), LVCMOS25_4mA_SLEW-ON_GPIO_O (Output), LVCMOS25_4mA_SLEW-OFF_GPIO_O (Output), LVCMOS25_6mA_SLEW-ON_GPIO_O (Output), LVCMOS25_6mA_SLEW-OFF_GPIO_O (Output), LVCMOS25_12mA_SLEW-ON_GPIO_O (Output), LVCMOS25_12mA_SLEW-OFF_GPIO_O (Output), LVCMOS25_16mA_SLEW-ON_GPIO_O (Output), LVCMOS25_16mA_SLEW-OFF_GPIO_O (Output), LVCMOS18_8mA_SLEW-OFF_GPIO_O (Output), LVCMOS18_2mA_SLEW-OFF_GPIO_O (Output), LVCMOS18_4mA_SLEW-OFF_GPIO_O (Output), LVCMOS18_6mA_SLEW-OFF_GPIO_O (Output), LVCMOS18_10mA_SLEW-OFF_GPIO_O (Output), LVCMOS18_12mA_SLEW-OFF_GPIO_O (Output), LVCMOS15_8mA_SLEW-OFF_GPIO_O (Output), LVCMOS15_2mA_SLEW-OFF_GPIO_O (Output), LVCMOS15_4mA_SLEW-OFF_GPIO_O (Output), LVCMOS15_6mA_SLEW-OFF_GPIO_O (Output), LVCMOS15_10mA_SLEW-OFF_GPIO_O (Output), LVCMOS12_8mA_SLEW-OFF_GPIO_O (Output), LVCMOS12_2mA_SLEW-OFF_GPIO_O (Output), LVCMOS12_4mA_SLEW-OFF_GPIO_O (Output), LVCMOS12_6mA_SLEW-OFF_GPIO_O (Output), SSTL25_C1_80ohm_SLEW-OFF_GPIO_O (Output), SSTL25_C1_120ohm_SLEW-OFF_GPIO_O (Output), SSTL25_C1_60ohm_SLEW-OFF_GPIO_O (Output), SSTL25_C1_48ohm_SLEW-OFF_GPIO_O (Output), SSTL25_C2_48ohm_SLEW-OFF_GPIO_O (Output), SSTL25_C2_60ohm_SLEW-OFF_GPIO_O (Output), SSTL25_C2_40ohm_SLEW-OFF_GPIO_O (Output), SSTL25_C2_34ohm_SLEW-OFF_GPIO_O (Output), SSTL18_C1_60ohm_SLEW-OFF_GPIO_O (Output), SSTL18_C1_80ohm_SLEW-OFF_GPIO_O (Output), SSTL18_C1_48ohm_SLEW-OFF_GPIO_O (Output), SSTL18_C1_40ohm_SLEW-OFF_GPIO_O (Output), SSTL18_C2_40ohm_SLEW-OFF_GPIO_O (Output), SSTL18_C2_48ohm_SLEW-OFF_GPIO_O (Output), SSTL18_C2_34ohm_SLEW-OFF_GPIO_O (Output), SSTL18_C2_30ohm_SLEW-OFF_GPIO_O (Output), SSTL15_C1_40ohm_SLEW-OFF_GPIO_O (Output), SSTL15_C1_48ohm_SLEW-OFF_GPIO_O (Output), SSTL15_C2_34ohm_SLEW-OFF_GPIO_O (Output), SSTL15_C2_30ohm_SLEW-OFF_GPIO_O (Output), SSTL15_C2_27ohm_SLEW-OFF_GPIO_O (Output), HSUL18_C1_55ohm_SLEW-OFF_GPIO_O (Output), HSUL18_C1_60ohm_SLEW-OFF_GPIO_O (Output), HSUL18_C1_40ohm_SLEW-OFF_GPIO_O (Output), HSUL18_C1_34ohm_SLEW-OFF_GPIO_O (Output), HSUL18_C2_25ohm_SLEW-OFF_GPIO_O (Output), HSUL18_C2_30ohm_SLEW-OFF_GPIO_O (Output), HSUL18_C2_27ohm_SLEW-OFF_GPIO_O (Output), HSUL18_C2_22ohm_SLEW-OFF_GPIO_O (Output), HSTL15_C1_50ohm_SLEW-OFF_GPIO_O (Output), HSTL15_C1_60ohm_SLEW-OFF_GPIO_O (Output), HSTL15_C1_40ohm_SLEW-OFF_GPIO_O (Output), HSTL15_C1_34ohm_SLEW-OFF_GPIO_O (Output), HSTL15_C2_25ohm_SLEW-OFF_GPIO_O (Output), HSTL15_C2_30ohm_SLEW-OFF_GPIO_O (Output), HSTL15_C2_27ohm_SLEW-OFF_GPIO_O (Output), HSTL15_C2_22ohm_SLEW-OFF_GPIO_O (Output), LVDS33_6mA_SLEW-OFF_GPIO_O (Output), LVDS33_4mA_SLEW-OFF_GPIO_O (Output), LVDS33_3P5mA_SLEW-OFF_GPIO_O (Output), LVDS33_3mA_SLEW-OFF_GPIO_O (Output)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
